(* Logix 5000 AddOnInstructionDefinition export Banner_TL70Pro_Param_v4; software revision 33.00 *)

TYPE Banner_IOL_Port_v4 :   // UDT that has all of the data items necessary to communicate with a specific Port on a IO-Link Master
STRUCT
   Port_Controlled : INT;   // Each bit represents a port on an IO-Link Master. Set to 1 to tell AOI to control that port.
   Port_Activate : INT;   // Each bit represents a port on an IO-Link Master. When ON that port will process any commands in queue.
   Port_Read : INT;   // Each bit represents a port on an IO-Link Master. Used to determine when device AOI has requested a Read command.
   Port_Write : INT;   // Each bit represents a port on an IO-Link Master. Used to determine when device AOI has requested a Write command.
   Port_RW_Complete : INT;   // Each bit represents a port on an IO-Link Master. Tells device AOI that Read or Write request has been completed.
   Port_Device_Read : INT;
   Data_Transfer : SINT[190];   // Array to transfer data from IO-Master to device AOIs.
END_STRUCT
END_TYPE

TYPE Banner_TL70Pro_Basic_SP_v4 :   // Basic parameters for a TL70 Pro segment.
STRUCT
   Basic_Color : SINT;   // 0 = Green, 1 = Red, 2 = Orange, 3 = Amber, 4 = Yellow, 5 = Lime Green, 6 = Spring Green, 7 = Cyan, 8 = Sky Blue, 9 = Blue, 10 = Violet, 11 = Magenta, 12 = Rose, 13 = White, 14 = Custom, 15 = Custom 2
   Basic_Flash_Rate : SINT;   // 0 = Medium, 1 = Fast, 2 = Slow, 3 = Custom Flash Rate
   Animation : SINT;   // 0 = Off, 1 = Steady, 2 = Flash, 3 = Two Color, 4 = Half/Half, 5 = Half/Half Rotate, 6 = Chase, 7 = Intesnity Sweep
   Color_1 : INT;   // 0 = Green, 1 = Red, 2 = Orange, 3 = Amber, 4 = Yellow, 5 = Lime Green, 6 = Spring Green, 7 = Cyan, 8 = Sky Blue, 9 = Blue, 10 = Violet, 11 = Magenta, 12 = Rose, 13 = White, 14 = Custom, 15 = Custom 2
   Color_1_Intensity : SINT;   // 0 = High, 1 = Low, 2 = Medium, 3 = Off, 4 = Custom
   Speed : SINT;   // 0 = Medium, 1 = Fast, 2 = Slow, 3 = Custom
   Pulse_Pattern : SINT;   // 0 = Normal, 1 = Strobe, 2 = Three Pulse, 3 = SOS, 4 = Random
   Color_2 : SINT;   // 0 = Green, 1 = Red, 2 = Orange, 3 = Amber, 4 = Yellow, 5 = Lime Green, 6 = Spring Green, 7 = Cyan, 8 = Sky Blue, 9 = Blue, 10 = Violet, 11 = Magenta, 12 = Rose, 13 = White, 14 = Custom, 15 = Custom 2
   Color_2_Intensity : SINT;   // 0 = High, 1 = Low, 2 = Medium, 3 = Off, 4 = Custom
END_STRUCT
END_TYPE

TYPE Banner_TL70Pro_Gauge_Center_Settings_v4 :   // TL70 Pro. BG = Background
STRUCT
   Percent_Width_of_Main_Segment : SINT;   // 1 to 100
   Main_Animation : INT;   // 0 = Off, 1 = Steady, 2 = Flash, 3 = Two Color Flash, 4 = Two Color Shift, 5 = Scroll, 6 = Center Scroll, 7 = Bounce, 8 = Center Bounce, 9 = Intensity Sweep, 10 = Two Color Sweep, 11 = Spectrum, 12 = Single End Steady, 13 = Single End Flash
   Main_Color_1 : INT;   // 0 = Green, 1 = Red, 2 = Orange, 3 = Amber, 4 = Yellow, 5 = Lime Green, 6 = Spring Green, 7 = Cyan, 8 = Sky Blue, 9 = Blue, 10 = Violet, 11 = Magenta, 12 = Rose, 13 = White, 14 = Custom, 15 = Custom 2
   Main_Color_1_Intensity : SINT;   // 0 = High, 1 = Low, 2 = Medium, 3 = Off, 4 = Custom
   Main_Speed : SINT;   // 0 = Medium, 1 = Fast, 2 = Slow, 3 = Custom Flash Rate
   Main_Pulse_Pattern : SINT;   // 0 = Normal, 1 = Strobe, 2 = Three Pulse, 3 = SOS, 4 = Random
   Main_Color_2 : INT;   // 0 = Green, 1 = Red, 2 = Orange, 3 = Amber, 4 = Yellow, 5 = Lime Green, 6 = Spring Green, 7 = Cyan, 8 = Sky Blue, 9 = Blue, 10 = Violet, 11 = Magenta, 12 = Rose, 13 = White, 14 = Custom, 15 = Custom 2
   Main_Color_2_Intensity : SINT;   // 0 = High, 1 = Low, 2 = Medium, 3 = Off, 4 = Custom
   Main_Scroll_Bounce_Style : SINT;   // 0 = Solid,1 = Tail, 2 = Ripple
   Main_Percent_Width_of_Color_1 : SINT;   // 0 to 100
   Main_Direction : SINT;   // 0 = Up, 1 = Down
   BG_Animation : INT;   // 0 = Off, 1 = Steady, 2 = Flash, 3 = Two Color Flash, 4 = Two Color Shift, 5 = Scroll, 6 = Center Scroll, 7 = Bounce, 8 = Center Bounce, 9 = Intensity Sweep, 10 = Two Color Sweep, 11 = Spectrum, 12 = Single End Steady, 13 = Single End Flash
   BG_Color_1 : INT;   // 0 = Green, 1 = Red, 2 = Orange, 3 = Amber, 4 = Yellow, 5 = Lime Green, 6 = Spring Green, 7 = Cyan, 8 = Sky Blue, 9 = Blue, 10 = Violet, 11 = Magenta, 12 = Rose, 13 = White, 14 = Custom, 15 = Custom 2
   BG_Color_1_Intensity : INT;   // 0 = High, 1 = Low, 2 = Medium, 3 = Off, 4 = Custom
   BG_Speed : SINT;   // 0 = Medium, 1 = Fast, 2 = Slow, 3 = Custom
   BG_Pulse_Pattern : SINT;   // 0 = Normal, 1 = Strobe, 2 = Three Pulse, 3 = SOS, 4 = Random
   BG_Color_2 : INT;   // 0 = Green, 1 = Red, 2 = Orange, 3 = Amber, 4 = Yellow, 5 = Lime Green, 6 = Spring Green, 7 = Cyan, 8 = Sky Blue, 9 = Blue, 10 = Violet, 11 = Magenta, 12 = Rose, 13 = White, 14 = Custom, 15 = Custom 2
   BG_Color_2_Intensity : SINT;   // 0 = High, 1 = Low, 2 = Medium, 3 = Off, 4 = Custom
   BG_Scroll_Bounce_Style : SINT;   // 0 = Solid, 1 = Tail, 2 = Ripple
   BG_Percent_Width_of_Color_1 : SINT;   // 1 to 100
   BG_Direction : SINT;   // 0 = Up, 1 = Down
END_STRUCT
END_TYPE

TYPE Banner_TL70Pro_Gauge_Mode_Config_v4 :
STRUCT
   Filtering : SINT;   // 0 = None, 1 = Low, 2 = Medium, 3 = High
   Hysteresis : SINT;   // 0 = None, 1 = Low, 2 = Medium, 3 = High
   Full_Scale_Value : INT;   // 0 to 100
END_STRUCT
END_TYPE

TYPE Banner_TL70Pro_Gauge_Threshold_Set_v4 :   // BG = Background
STRUCT
   Threshold_Enable : SINT;   // 0 = Threshold Disabled, 1 = Threshold Enabled
   Threshold_Value : SINT;   // 0 to 100 percent
   Threshold_Comparison : SINT;   // 0 = Less than or equal to, 1 = Greater than or equal to
   Percent_Width_of_Main_Segment : SINT;   // 0 to 100 percent
   Main_Animation : INT;   // 0 = Off, 1 = Steady, 2 = Flash, 3 = Two Color Flash, 4 = Two Color Shift, 5 = Scroll, 6 = Center Scroll, 7 = Bounce, 8 = Center Bounce, 9 = Intensity Sweep, 10 = Two Color Sweep, 11 = Spectrum, 12 = Single End Steady, 13 = Single End Flash
   Main_Color_1 : INT;   // 0 = Green, 1 = Red, 2 = Orange, 3 = Amber, 4 = Yellow, 5 = Lime Green, 6 = Spring Green, 7 = Cyan, 8 = Sky Blue, 9 = Blue, 10 = Violet, 11 = Magenta, 12 = Rose, 13 = White, 14 = Custom, 15 = Custom 2
   Main_Color_1_Intensity : SINT;   // 0 = High, 1= Low, 2 = Medium, 3 = Off, 4 = Custom
   Main_Speed : SINT;   // 0 = Medium, 1 = Fast, 2 = Slow, 3 = Custom Flash Rate
   Main_Pulse_Pattern : SINT;   // 0 = Normal, 1 = Strobe, 2 = Three Pulse, 3 = SOS, 4 = Random
   Main_Color_2 : INT;   // 0 = Green, 1 = Red, 2 = Orange, 3 = Amber, 4 = Yellow, 5 = Lime Green, 6 = Spring Green, 7 = Cyan, 8 = Sky Blue, 9 = Blue, 10 = Violet, 11 = Magenta, 12 = Rose, 13 = White, 14 = Custom, 15 = Custom 2
   Main_Color_2_Intensity : SINT;   // 0 = High,1 = Low, 2= Medium, 3 = Off, 4 = Custom
   Main_Scroll_Bounce_Style : SINT;   // 0 = Solid, 1 = Tail, 2 = Ripple
   Main_Percent_Width_of_Color_1 : SINT;   // 1 to 100 percent
   Main_Direction : SINT;   // 0 = Up, 1 = Down
   BG_Animation : INT;   // 0 = Off, 1 = Steady, 2 = Flash, 3 = Two Color Flash, 4 = Two Color Shift, 5 = Scroll, 6 = Center Scroll, 7 = Bounce, 8 = Center Bounce, 9 = Intensity Sweep, 10 = Two Color Sweep, 11 = Spectrum, 12 = Single End Steady, 13 = Single End Flash
   BG_Color_1 : INT;   // 0 = Green, 1 = Red, 2 = Orange, 3 = Amber, 4 = Yellow, 5 = Lime Green, 6 = Spring Green, 7 = Cyan, 8 = Sky Blue, 9 = Blue, 10 = Violet, 11 = Magenta, 12 = Rose, 13 = White, 14 = Custom, 15 = Custom 2
   BG_Color_1_Intensity : SINT;   // 0 = High, 1 = Low, 2 = Medium, 3 = Off, 4 = Custom
   BG_Speed : SINT;   // 0 = Medium, 1 = Fast, 2 = Slow, 3 = Custom Flash Rate
   BG_Pulse_Pattern : SINT;   // 0 = Normal, 1 = Strobe, 2 = Three Pulse, 3 = SOS, 4 = Random
   BG_Color_2 : INT;   // 0 = Green, 1 = Red, 2 = Orange, 3 = Amber, 4 = Yellow, 5 = Lime Green, 6 = Spring Green, 7 = Cyan, 8 = Sky Blue, 9 = Blue, 10 = Violet, 11 = Magenta, 12 = Rose, 13 = White, 14 = Custom, 15 = Custom 2
   BG_Color_2_Intensity : SINT;   // 0 = High, 1 = Low, 2 = Medium, 3 = Off, 4 = Custom
   BG_Scroll_Bounce_Style : SINT;   // 0 = Solid, 1 = Tail, 2 = Ripple
   BG_Percent_Width_of_Color_1 : SINT;   // 1 to 100
   BG_Direction : SINT;   // 0 = Up, 1 = Down
END_STRUCT
END_TYPE

TYPE Banner_TL70Pro_General_Level_Config_v4 :
STRUCT
   BG_Color : SINT;   // Background Color. 0 = Green, 1 = Red, 2 = Orange, 3 = Amber, 4 = Yellow, 5 = Lime Green, 6 = Spring Green, 7 = Cyan, 8 = Sky Blue, 9 = Blue, 10 = Violet, 11 = Magenta, 12 = Rose, 13 = White, 14 = Custom, 15 = Custom 2.
   BG_Intensity : SINT;   // 0 = High, 1 = Low, 2 = Medium, 3 = Off, 4 = Custom
   Dominance : SINT;   // 0 = Non-Dominant, 1 = Dominant
   Sub_Segment_Style : SINT;   // 0 = Solid, 1 = Analog
   Filtering : SINT;   // 0 = None, 1 = Low, 2 = Medium, 3 = High
   Hysteresis : SINT;   // 0 = None, 1 = Low, 2 = Medium, 3 = High
   Full_Scale_Value : INT;
END_STRUCT
END_TYPE

TYPE Banner_TL70Pro_General_Seg_Config_v4 :
STRUCT
   Background_Color : INT;   // 0 = Green, 1 = Red, 2 = Orange, 3 = Amber, 4 = Yellow, 5 = Lime Green, 6 = Spring Green, 7 = Cyan, 8 = Sky Blue, 9 = Blue, 10 = Violet, 11 = Magenta, 12 = Rose, 13 = White, 14 = Custom, 15 = Custom 2
   Background_Intensity : SINT;   // 0 = High, 1 = Low, 2 = Medium, 3 = Off, 4 = Custom
   Animation_Synchro : SINT;   // 0 = Animation Sync Disabled, 1 = Animation Sync Enabled
END_STRUCT
END_TYPE

TYPE Banner_TL70Pro_Level_Base_Config_v4 :
STRUCT
   Animation : INT;   // 0 = Off, 1 = Steady, 2 = Flash, 3 = Two Color Flash, 4 = Two Color Shift, 5 = Scroll, 6 = Center Scroll, 7 = Bounce, 8 = Center Bounce, 9 = Intensity Sweep, 10 = Two Color Sweep, 11 = Spectrum, 12 = Single End Steady, 13 = Daylight White, 14 = Custom 1, 15 = Custom 2
   Color_1 : INT;   // 0 = Green, 1 = Red, 2 = Orange, 3 = Amber, 4 = Yellow, 5 = Lime Green, 6 = Spring Green, 7 = Cyan, 8 = Sky Blue, 9 = Blue, 10 = Violet, 11 = Magenta, 12 = Rose, 13 = White, 14 = Custom, 15 = Custom 2
   Color_1_Intensity : SINT;   // 0 = High, 1 = Low, 2 = Medium, 3 = Off, 4 = Custom
   Speed : SINT;   // 0 = Medium, 1 = Fast, 2 = Slow, 3 = Custom Flash Rate
   Pulse_Pattern : SINT;   // 0 = Normal, 1 = Strobe, 2 = Three Pulse, 3 = SOS, 4 = Random
   Color_2 : INT;   // 0 = Green, 1 = Red, 2 = Orange, 3 = Amber, 4 = Yellow, 5 = Lime Green, 6 = Spring Green, 7 = Cyan, 8 = Sky Blue, 9 = Blue, 10 = Violet, 11 = Magenta, 12 = Rose, 13 = White, 14 = Custom, 15 = Custom 2
   Color_2_Intensity : INT;   // 0 = High, 1 = Low, 2 = Medium, 3 = Off, 4 = Custom
   Scroll_Bounce_Style : SINT;   // 0 = Solid, 1 = Tail, 2 = Ripple
   Percent_Width_of_Color_1 : SINT;   // 0 to 100. The size of the scrolling segement
   Direction : SINT;   // 0 = Up, 1 = Down
END_STRUCT
END_TYPE

TYPE Banner_TL70Pro_RD_v4 :   // UDT that stores the Read Data for a TL70 Pro.
STRUCT
   Master_Cycle_Time : INT;
   Min_Cycle_Time : INT;
   M_Sequence_Capability : INT;
   IO_Link_Version_ID : INT;
   Process_Data_Input_Length : INT;
   Process_Data_Output_Length : INT;
   Combined_Vendor_ID : DINT;   // IO-Link Vendor ID
   Vendor_ID1 : INT;
   Vendor_ID2 : INT;
   Combined_Device_ID : DINT;   // IO-Link Device ID
   Device_ID1 : INT;
   Device_ID2 : INT;
   Device_ID3 : INT;
   Serial_Number : STRING;
END_STRUCT
END_TYPE

TYPE Banner_TL70Pro_Threshold_Config_v4 :
STRUCT
   Threshold_Enable : SINT;   // 0 = Threshold Disabled, 1 = Threshold Enabled
   Threshold_Value_Percent : SINT;   // 0 to 100 percent.
   Threshold_Comparison : SINT;   // 0 = Less than or equal to, 1 = Greater than or equal to
   Threshold_Override : SINT;   // 0 = Override not enabled, 1 = Override Enabled
   Animation : INT;   // 0 = Off, 1 = Steady, 2 = Flash, 3 = Two Color Flash, 4 = Two Color Shift, 5 = Scroll, 6 = Center Scroll, 7 = Bounce, 8 = Center Bounce, 9 = Intensity Sweep, 10 = Two Color Sweep, 11 = Spectrum, 12 = Single End Steady, 13 = Single End Flash
   Color_1 : INT;   // 0 = Green, 1 = Red, 2 = Orange, 3 = Amber, 4 = Yellow, 5 = Lime Green, 6 = Spring Green, 7 = Cyan, 8 = Sky Blue, 9 = Blue, 10 = Violet, 11 = Magenta, 12 = Rose, 13 = White, 14 = Custom, 15 = Custom 2
   Color_1_Intensity : SINT;   // 0 = High, 1 = Low, 2 = Medium, 3 = Off, 4 = Custom
   Speed : SINT;   // 0 = Medium, 1 = Fast, 2 = Slow, 3 = Custom Flash Rate
   Pulse_Pattern : SINT;   // 0 = Normal, 1 = Strobe, 2 = Three Pulse, 3 = SOS, 4 = Random
   Color_2 : INT;   // 0 = Green, 1 = Red, 2 = Orange, 3 = Amber, 4 = Yellow, 5 = Lime Green, 6 = Spring Green, 7 = Cyan, 8 = Sky Blue, 9 = Blue, 10 = Violet, 11 = Magenta, 12 = Rose, 13 = White, 14 = Custom, 15 = Custom 2
   Color_2_Intensity : SINT;   // 0 = High, 1 = Low, 2 = Medium, 3 = Off, 4 = Custom
   Scroll_Bounce_Style : SINT;   // 0 = Solid, 1 = Tail, 2 = Ripple
   Percent_Width_of_Color_1 : SINT;   // 0 to 100
   Direction : SINT;   // 0 = Up, 1 = Down
END_STRUCT
END_TYPE

TYPE Banner_TL70Pro_v4 :   // All of the parameters for a TL70 Pro.
STRUCT
   Initial_Global_Read : BOOL;   // Determines if all of the IO-Link data has been read into the PLC yet
   Command : INT;   // Value placed in here will activate a read or write to a specifc IO-Link Index
   Read : Banner_TL70Pro_RD_v4;   // Read Only Data
   Write : Banner_TL70Pro_WD_v4;   // Write Data
   Archive : Banner_TL70Pro_WD_v4;   // Archive of the Write Data
   Reset : BOOL;   // Resets AOI. This will force a complete parameter read of the sensor.
END_STRUCT
END_TYPE

TYPE Banner_TL70Pro_WD_v4 :   // UDT that stores the Write Data for a TL70 Pro.
STRUCT
   System_Command : INT;   // See IODD file for list of commands that can be activated via the System Command interface
   Parameter_Access_Lock : SINT;   // Write access to all parameters is prohibited while value is 1. Only this parameter can be adjusted when value is 1.
   Data_Storage_Lock : SINT;   // Automatic data storage is disabled when this value is equal to 1. Read access is not affected.
   Local_Parameterization_Lock : SINT;   // Parameterization via local control elements on device is disabled.
   Local_User_Interface_Lock : SINT;   // Operation of local user interface is disabled.
   Operating_Mode_Selection : SINT;   // 0 = Basic Mode, 1 = Run Mode, 2 = Level Mode, 3 = Gauge Mode, 4 = Advance Mode
   General_Segment_Config : Banner_TL70Pro_General_Seg_Config_v4;
   Segment_Config : Banner_TL70Pro_Basic_SP_v4[7];
   General_Level_Config : Banner_TL70Pro_General_Level_Config_v4;
   Level_Base_Config : Banner_TL70Pro_Level_Base_Config_v4;
   Level_Threshold_Config : Banner_TL70Pro_Threshold_Config_v4[5];
   Custom_1_Red : INT;   // 0 to 255. Value of the Red portion of the RGB color value for Custom 1
   Custom_1_Green : INT;   // 0 to 255. Value of the Green portion of the RGB color value for Custom 1.
   Custom_1_Blue : INT;   // 0 to 255. Value of the Blue portion of the RGB color value for Custom 1.
   Custom_2_Red : INT;   // 0 to 255. Value of the Red portion of the RGB color value for Custom 2.
   Custom_2_Green : INT;   // 0 to 255. Value of the Green portion of the RGB color value for Custom 2.
   Custom_2_Blue : INT;   // 0 to 255. Value of the Blue portion of the RGB color value for Custom 2.
   Orientation : SINT;   // 0 = Standard, 1 = Inverted
   Custom_Intensity : SINT;   // 0 to 100
   Custom_Frequency : INT;   // 0 to 255
   Gauge_Mode_Config : Banner_TL70Pro_Gauge_Mode_Config_v4;
   Gauge_Mode_Center : Banner_TL70Pro_Gauge_Center_Settings_v4;
   Gauge_Mode_Threshold : Banner_TL70Pro_Gauge_Threshold_Set_v4[3];
   Advanced_Audible_Type : SINT;   // 0 = Beep, 1 = Sweep, 2 = Tone
   Sweep_Type : SINT;   // 0 = Up, 1 = Down, 2 = Up Down, 3 = Down Up
   Frequency_1 : SINT;   // 0 = Off, 1 = Low, 2 = Standard, 3 = High
   Frequency_2 : SINT;   // 0 = Off, 1 = Low, 2 = Standard, 3 = High
END_STRUCT
END_TYPE

ADD_ON_INSTRUCTION Banner_TL70Pro_Param_v4   (* revision 4.1, vendor Banner Engineering *)
// AOI to read and write parameter data to an IO-Link TL70 Pro.
VAR_IN_OUT
   TL70Pro : Banner_TL70Pro_v4; {required}
   Port_Data : Banner_IOL_Port_v4; {required}
END_VAR
VAR_INPUT
   Port : INT; {required}   // Port Number that device is plugged into.
END_VAR
VAR
   Local_Control : DINT; {access None}
   Global_Read_Command_Value : INT; {access None}
   Global_Write_Command_Value : INT; {access None}
   Command_Being_Processed : BOOL; {access None}
   Update_Archive : BOOL; {access None}
   Index_Write_Inprocess : DINT; {access None}
   Index_Write_Control : DINT; {access None}
   Inprocess_Index : DINT; {access None}
   Index_R : DINT; {access None}
   BS_Index : DINT; {access None}
   Index_W : DINT; {access None}
   W_Index : DINT; {access None}
   Index_Segment_Read : DINT; {access None}
   GT_Index2 : DINT; {access None}
   GT_Index1 : DINT; {access None}
   LT_Index2 : DINT; {access None}
   LT_Index1 : DINT; {access None}
END_VAR

ROUTINE Logic   (* ladder *)
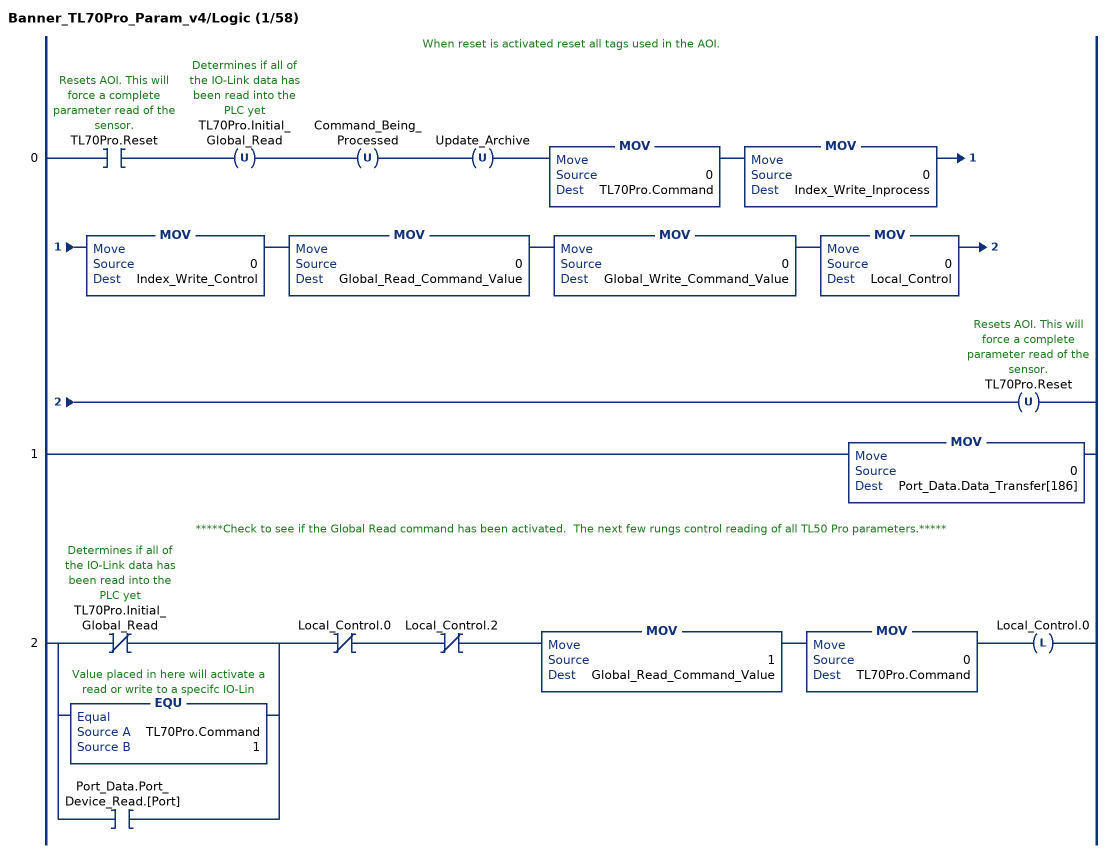
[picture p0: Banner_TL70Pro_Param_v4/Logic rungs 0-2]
   // When reset is activated reset all tags used in the AOI.
   0: XIC(TL70Pro.Reset)OTU(TL70Pro.Initial_Global_Read)OTU(Command_Being_Processed)OTU(Update_Archive)MOV(0,TL70Pro.Command)MOV(0,Index_Write_Inprocess)MOV(0,Index_Write_Control)MOV(0,Global_Read_Command_Value)MOV(0,Global_Write_Command_Value)MOV(0,Local_Control)OTU(TL70Pro.Reset);
   1: MOV(0,Port_Data.Data_Transfer[186]);
   // *****Check to see if the Global Read command has been activated.  The next few rungs control reading of all TL50 Pro parameters.*****
   2: [XIO(TL70Pro.Initial_Global_Read) ,EQU(TL70Pro.Command,1) ,XIC(Port_Data.Port_Device_Read.[Port]) ]XIO(Local_Control.0)XIO(Local_Control.2)MOV(1,Global_Read_Command_Value)MOV(0,TL70Pro.Command)OTL(Local_Control.0);
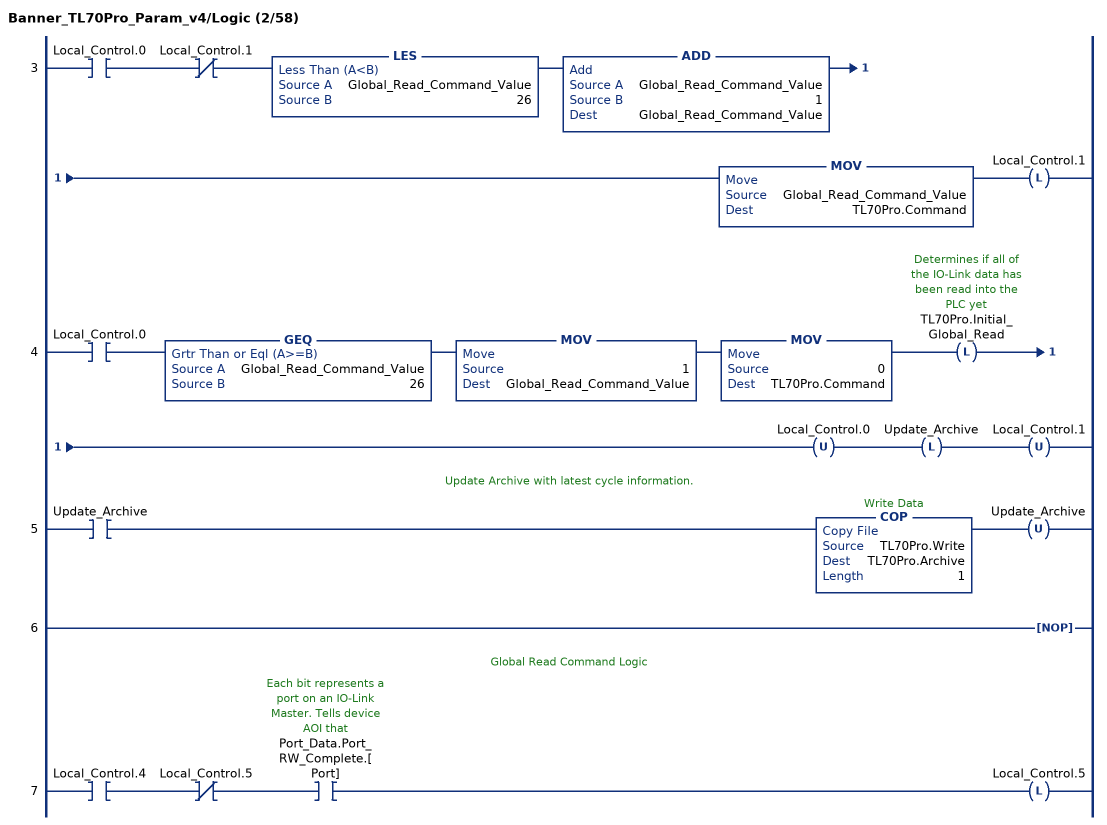
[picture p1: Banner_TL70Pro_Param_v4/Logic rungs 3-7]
   3: XIC(Local_Control.0)XIO(Local_Control.1)LES(Global_Read_Command_Value,26)ADD(Global_Read_Command_Value,1,Global_Read_Command_Value)MOV(Global_Read_Command_Value,TL70Pro.Command)OTL(Local_Control.1);
   4: XIC(Local_Control.0)GEQ(Global_Read_Command_Value,26)MOV(1,Global_Read_Command_Value)MOV(0,TL70Pro.Command)OTL(TL70Pro.Initial_Global_Read)OTU(Local_Control.0)OTL(Update_Archive)OTU(Local_Control.1);
   // Update Archive with latest cycle information.
   5: XIC(Update_Archive)COP(TL70Pro.Write,TL70Pro.Archive,1)OTU(Update_Archive);
   6: NOP();
   // Global Read Command Logic
   7: XIC(Local_Control.4)XIO(Local_Control.5)XIC(Port_Data.Port_RW_Complete.[Port])OTL(Local_Control.5);
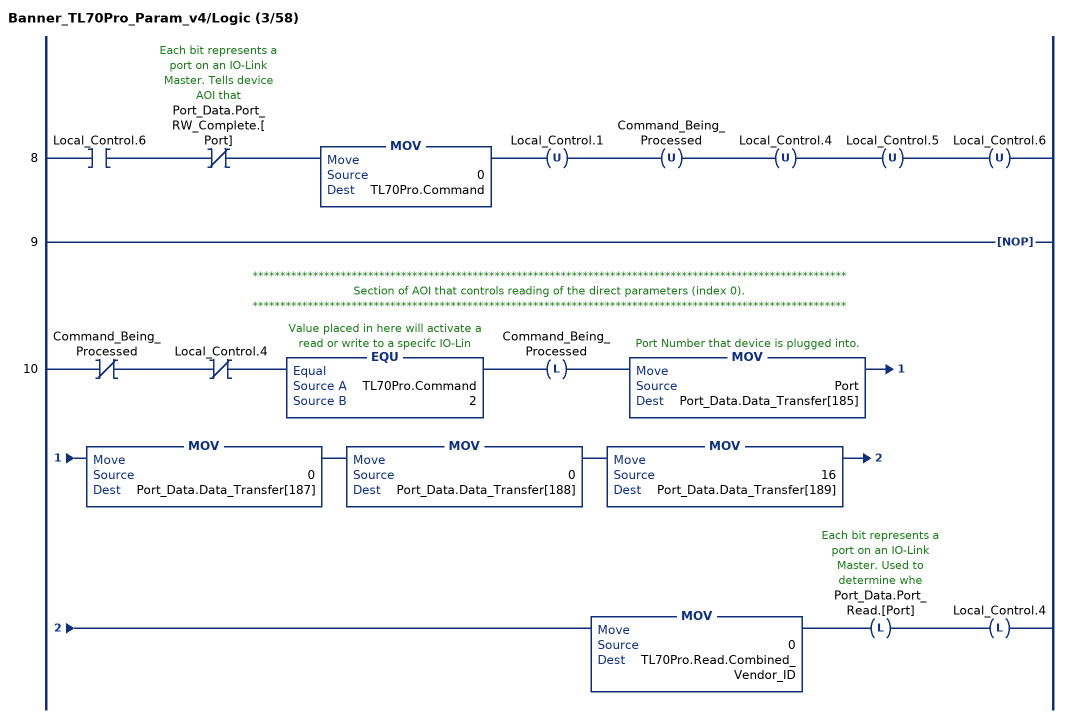
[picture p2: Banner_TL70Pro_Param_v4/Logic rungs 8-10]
   8: XIC(Local_Control.6)XIO(Port_Data.Port_RW_Complete.[Port])MOV(0,TL70Pro.Command)OTU(Local_Control.1)OTU(Command_Being_Processed)OTU(Local_Control.4)OTU(Local_Control.5)OTU(Local_Control.6);
   9: NOP();
   // ************************************************************************************************************
   // Section of AOI that controls reading of the direct parameters (index 0).
   // ************************************************************************************************************
   10: XIO(Command_Being_Processed)XIO(Local_Control.4)EQU(TL70Pro.Command,2)OTL(Command_Being_Processed)MOV(Port,Port_Data.Data_Transfer[185])MOV(0,Port_Data.Data_Transfer[187])MOV(0,Port_Data.Data_Transfer[188])MOV(16,Port_Data.Data_Transfer[189])MOV(0,TL70Pro.Read.Combined_Vendor_ID)OTL(Port_Data.Port_Read.[Port])OTL(Local_Control.4);
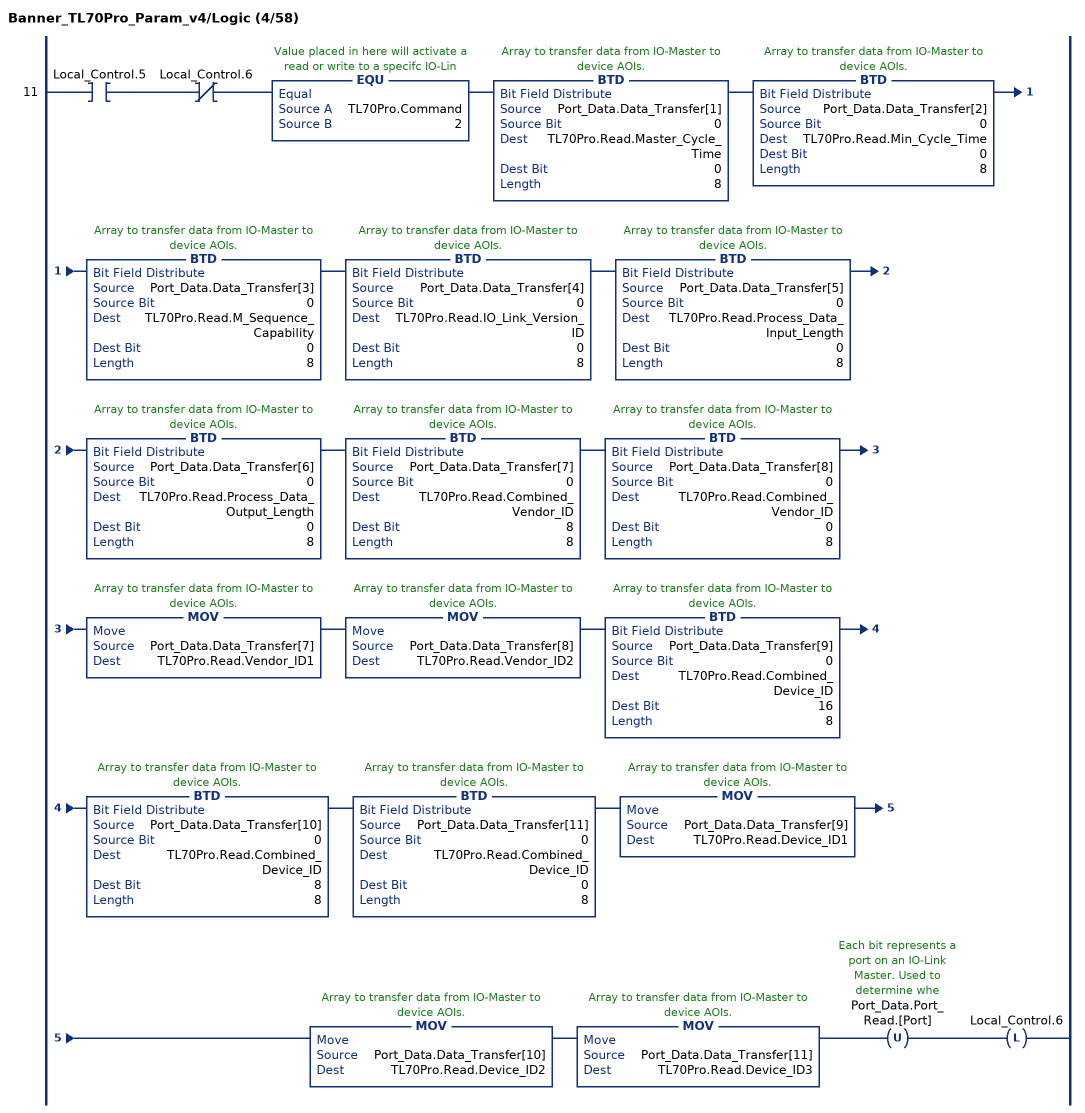
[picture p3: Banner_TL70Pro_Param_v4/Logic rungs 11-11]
   11: XIC(Local_Control.5)XIO(Local_Control.6)EQU(TL70Pro.Command,2)BTD(Port_Data.Data_Transfer[1],0,TL70Pro.Read.Master_Cycle_Time,0,8)BTD(Port_Data.Data_Transfer[2],0,TL70Pro.Read.Min_Cycle_Time,0,8)BTD(Port_Data.Data_Transfer[3],0,TL70Pro.Read.M_Sequence_Capability,0,8)BTD(Port_Data.Data_Transfer[4],0,TL70Pro.Read.IO_Link_Version_ID,0,8)BTD(Port_Data.Data_Transfer[5],0,TL70Pro.Read.Process_Data_Input_Length,0,8)BTD(Port_Data.Data_Transfer[6],0,TL70Pro.Read.Process_Data_Output_Length,0,8)BTD(Port_Data.Data_Transfer[7],0,TL70Pro.Read.Combined_Vendor_ID,8,8)BTD(Port_Data.Data_Transfer[8],0,TL70Pro.Read.Combined_Vendor_ID,0,8)MOV(Port_Data.Data_Transfer[7],TL70Pro.Read.Vendor_ID1)MOV(Port_Data.Data_Transfer[8],TL70Pro.Read.Vendor_ID2)BTD(Port_Data.Data_Transfer[9],0,TL70Pro.Read.Combined_Device_ID,16,8)BTD(Port_Data.Data_Transfer[10],0,TL70Pro.Read.Combined_Device_ID,8,8)BTD(Port_Data.Data_Transfer[11],0,TL70Pro.Read.Combined_Device_ID,0,8)MOV(Port_Data.Data_Transfer[9],TL70Pro.Read.Device_ID1)MOV(Port_Data.Data_Transfer[10],TL70Pro.Read.Device_ID2)MOV(Port_Data.Data_Transfer[11],TL70Pro.Read.Device_ID3)OTU(Port_Data.Port_Read.[Port])OTL(Local_Control.6);
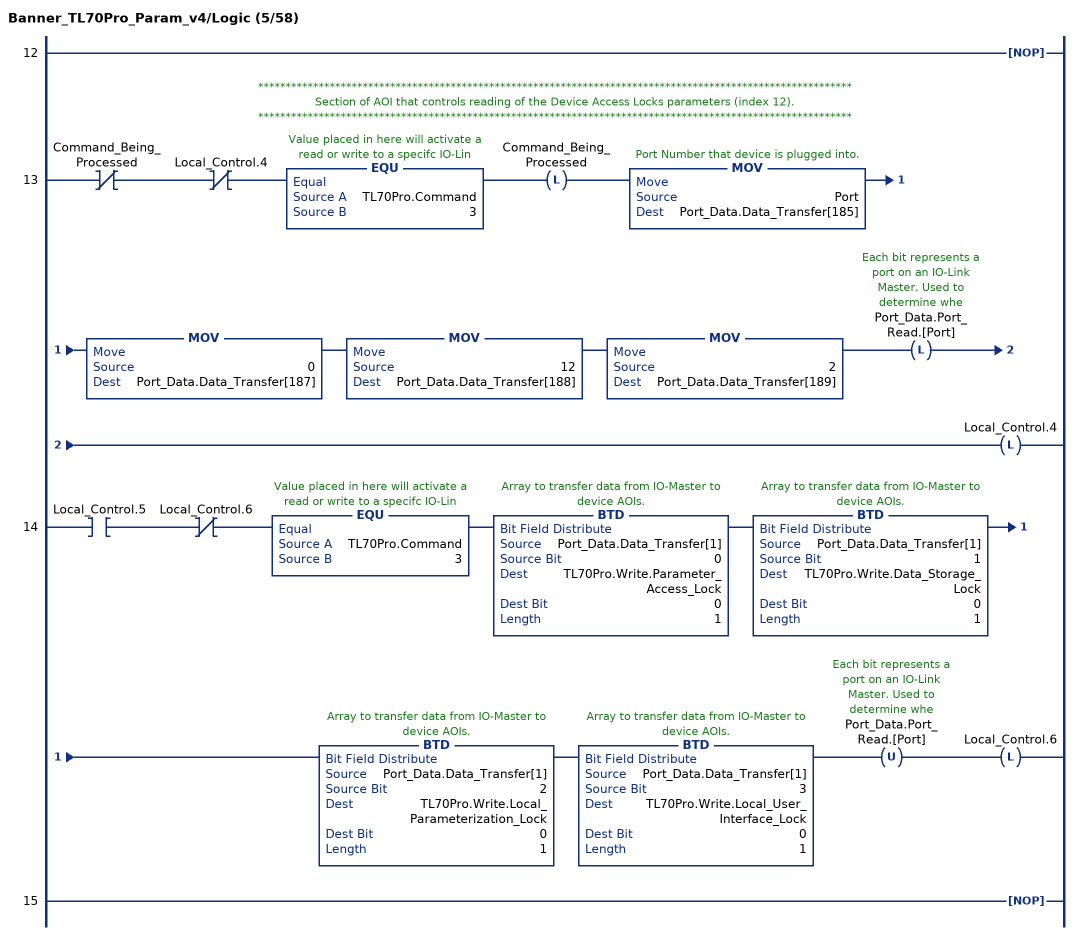
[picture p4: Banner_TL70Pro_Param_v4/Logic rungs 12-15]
   12: NOP();
   // ************************************************************************************************************
   // Section of AOI that controls reading of the Device Access Locks parameters (index 12).
   // ************************************************************************************************************
   13: XIO(Command_Being_Processed)XIO(Local_Control.4)EQU(TL70Pro.Command,3)OTL(Command_Being_Processed)MOV(Port,Port_Data.Data_Transfer[185])MOV(0,Port_Data.Data_Transfer[187])MOV(12,Port_Data.Data_Transfer[188])MOV(2,Port_Data.Data_Transfer[189])OTL(Port_Data.Port_Read.[Port])OTL(Local_Control.4);
   14: XIC(Local_Control.5)XIO(Local_Control.6)EQU(TL70Pro.Command,3)BTD(Port_Data.Data_Transfer[1],0,TL70Pro.Write.Parameter_Access_Lock,0,1)BTD(Port_Data.Data_Transfer[1],1,TL70Pro.Write.Data_Storage_Lock,0,1)BTD(Port_Data.Data_Transfer[1],2,TL70Pro.Write.Local_Parameterization_Lock,0,1)BTD(Port_Data.Data_Transfer[1],3,TL70Pro.Write.Local_User_Interface_Lock,0,1)OTU(Port_Data.Port_Read.[Port])OTL(Local_Control.6);
   15: NOP();
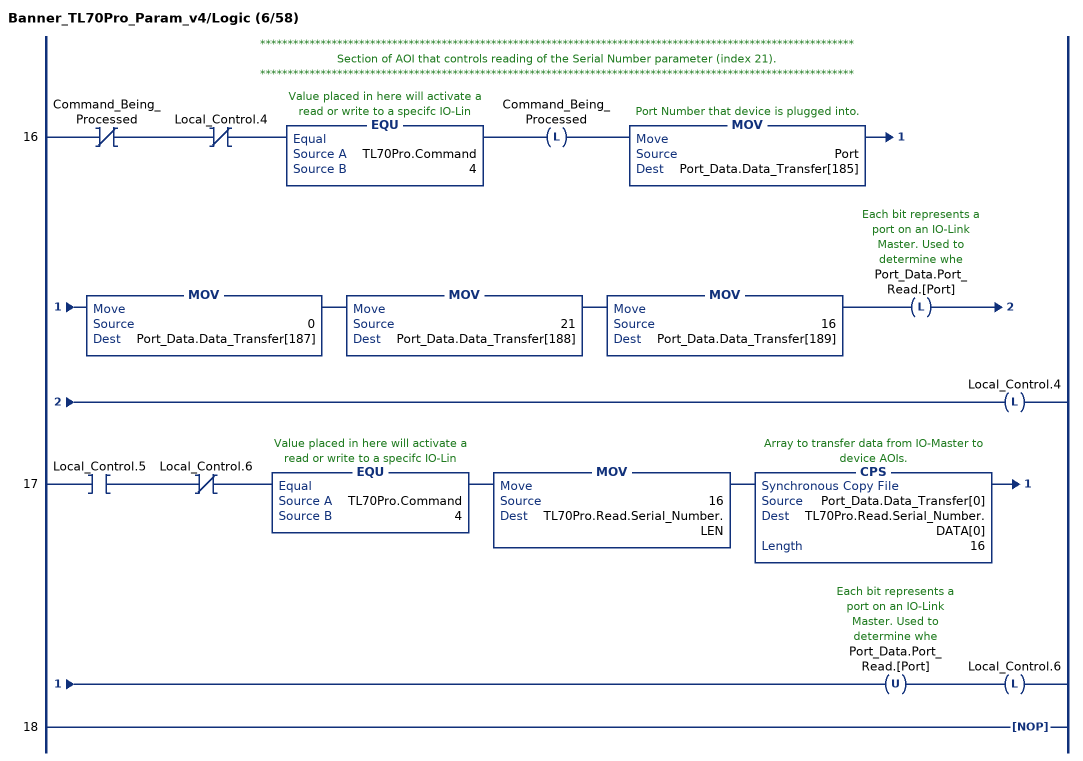
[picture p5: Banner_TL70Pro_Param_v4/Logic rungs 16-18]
   // ************************************************************************************************************
   // Section of AOI that controls reading of the Serial Number parameter (index 21).
   // ************************************************************************************************************
   16: XIO(Command_Being_Processed)XIO(Local_Control.4)EQU(TL70Pro.Command,4)OTL(Command_Being_Processed)MOV(Port,Port_Data.Data_Transfer[185])MOV(0,Port_Data.Data_Transfer[187])MOV(21,Port_Data.Data_Transfer[188])MOV(16,Port_Data.Data_Transfer[189])OTL(Port_Data.Port_Read.[Port])OTL(Local_Control.4);
   17: XIC(Local_Control.5)XIO(Local_Control.6)EQU(TL70Pro.Command,4)MOV(16,TL70Pro.Read.Serial_Number.LEN)CPS(Port_Data.Data_Transfer[0],TL70Pro.Read.Serial_Number.DATA[0],16)OTU(Port_Data.Port_Read.[Port])OTL(Local_Control.6);
   18: NOP();
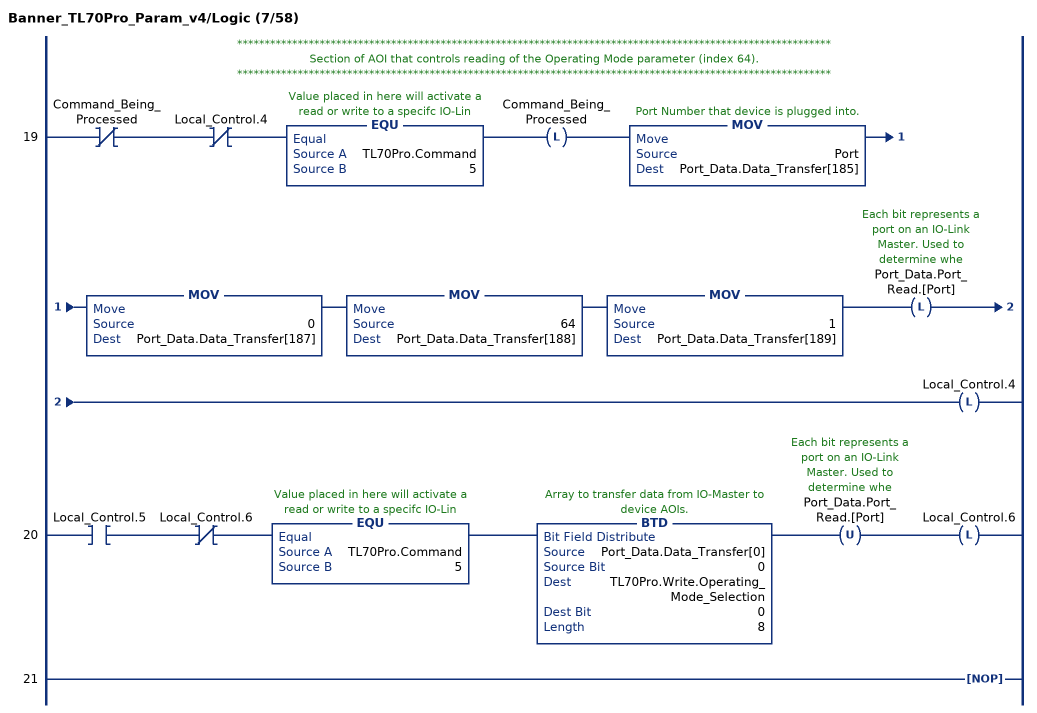
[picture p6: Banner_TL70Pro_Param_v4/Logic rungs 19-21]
   // ************************************************************************************************************
   // Section of AOI that controls reading of the Operating Mode parameter (index 64).
   // ************************************************************************************************************
   19: XIO(Command_Being_Processed)XIO(Local_Control.4)EQU(TL70Pro.Command,5)OTL(Command_Being_Processed)MOV(Port,Port_Data.Data_Transfer[185])MOV(0,Port_Data.Data_Transfer[187])MOV(64,Port_Data.Data_Transfer[188])MOV(1,Port_Data.Data_Transfer[189])OTL(Port_Data.Port_Read.[Port])OTL(Local_Control.4);
   20: XIC(Local_Control.5)XIO(Local_Control.6)EQU(TL70Pro.Command,5)BTD(Port_Data.Data_Transfer[0],0,TL70Pro.Write.Operating_Mode_Selection,0,8)OTU(Port_Data.Port_Read.[Port])OTL(Local_Control.6);
   21: NOP();
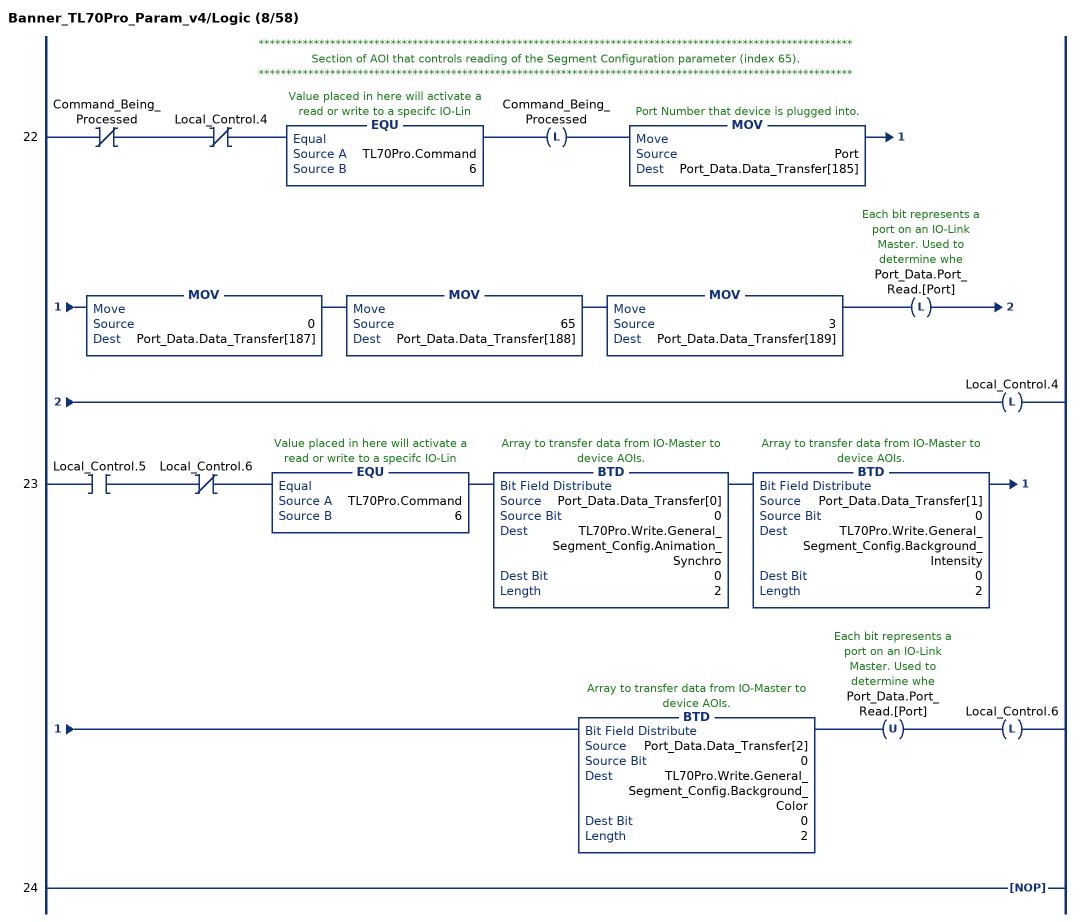
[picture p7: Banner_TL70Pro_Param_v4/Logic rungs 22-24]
   // ************************************************************************************************************
   // Section of AOI that controls reading of the Segment Configuration parameter (index 65).
   // ************************************************************************************************************
   22: XIO(Command_Being_Processed)XIO(Local_Control.4)EQU(TL70Pro.Command,6)OTL(Command_Being_Processed)MOV(Port,Port_Data.Data_Transfer[185])MOV(0,Port_Data.Data_Transfer[187])MOV(65,Port_Data.Data_Transfer[188])MOV(3,Port_Data.Data_Transfer[189])OTL(Port_Data.Port_Read.[Port])OTL(Local_Control.4);
   23: XIC(Local_Control.5)XIO(Local_Control.6)EQU(TL70Pro.Command,6)BTD(Port_Data.Data_Transfer[0],0,TL70Pro.Write.General_Segment_Config.Animation_Synchro,0,2)BTD(Port_Data.Data_Transfer[1],0,TL70Pro.Write.General_Segment_Config.Background_Intensity,0,2)BTD(Port_Data.Data_Transfer[2],0,TL70Pro.Write.General_Segment_Config.Background_Color,0,2)OTU(Port_Data.Port_Read.[Port])OTL(Local_Control.6);
   24: NOP();
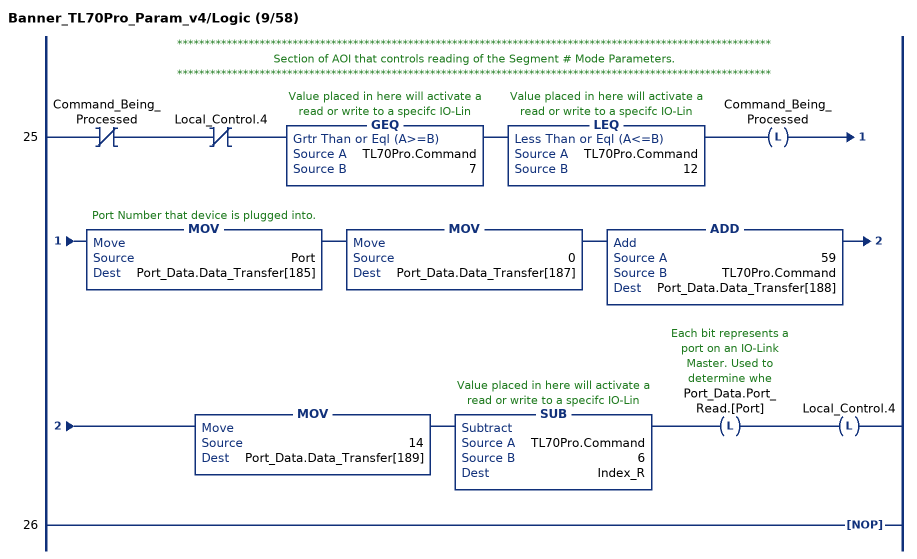
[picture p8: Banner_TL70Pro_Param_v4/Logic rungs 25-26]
   // ************************************************************************************************************
   // Section of AOI that controls reading of the Segment # Mode Parameters.
   // ************************************************************************************************************
   25: XIO(Command_Being_Processed)XIO(Local_Control.4)GEQ(TL70Pro.Command,7)LEQ(TL70Pro.Command,12)OTL(Command_Being_Processed)MOV(Port,Port_Data.Data_Transfer[185])MOV(0,Port_Data.Data_Transfer[187])ADD(59,TL70Pro.Command,Port_Data.Data_Transfer[188])MOV(14,Port_Data.Data_Transfer[189])SUB(TL70Pro.Command,6,Index_R)OTL(Port_Data.Port_Read.[Port])OTL(Local_Control.4);
   26: NOP();
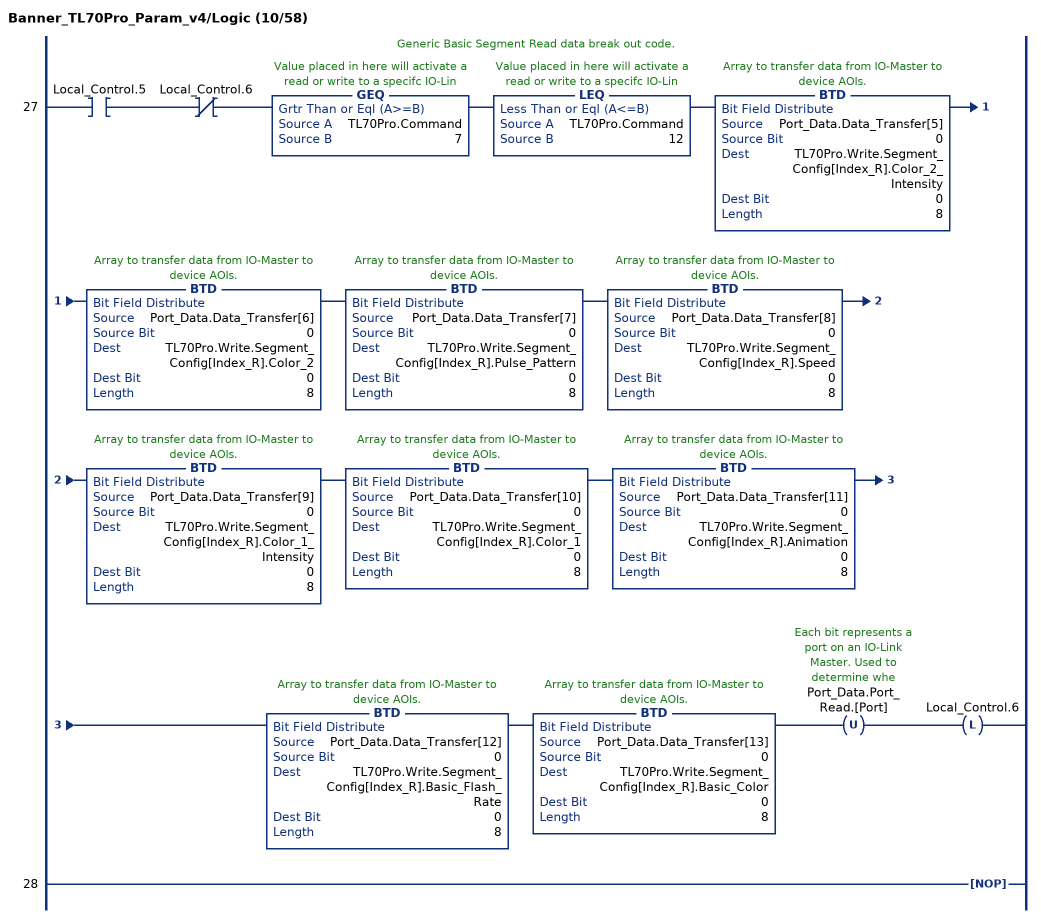
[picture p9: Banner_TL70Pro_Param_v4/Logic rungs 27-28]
   // Generic Basic Segment Read data break out code.
   27: XIC(Local_Control.5)XIO(Local_Control.6)GEQ(TL70Pro.Command,7)LEQ(TL70Pro.Command,12)BTD(Port_Data.Data_Transfer[5],0,TL70Pro.Write.Segment_Config[Index_R].Color_2_Intensity,0,8)BTD(Port_Data.Data_Transfer[6],0,TL70Pro.Write.Segment_Config[Index_R].Color_2,0,8)BTD(Port_Data.Data_Transfer[7],0,TL70Pro.Write.Segment_Config[Index_R].Pulse_Pattern,0,8)BTD(Port_Data.Data_Transfer[8],0,TL70Pro.Write.Segment_Config[Index_R].Speed,0,8)BTD(Port_Data.Data_Transfer[9],0,TL70Pro.Write.Segment_Config[Index_R].Color_1_Intensity,0,8)BTD(Port_Data.Data_Transfer[10],0,TL70Pro.Write.Segment_Config[Index_R].Color_1,0,8)BTD(Port_Data.Data_Transfer[11],0,TL70Pro.Write.Segment_Config[Index_R].Animation,0,8)BTD(Port_Data.Data_Transfer[12],0,TL70Pro.Write.Segment_Config[Index_R].Basic_Flash_Rate,0,8)BTD(Port_Data.Data_Transfer[13],0,TL70Pro.Write.Segment_Config[Index_R].Basic_Color,0,8)OTU(Port_Data.Port_Read.[Port])OTL(Local_Control.6);
   28: NOP();
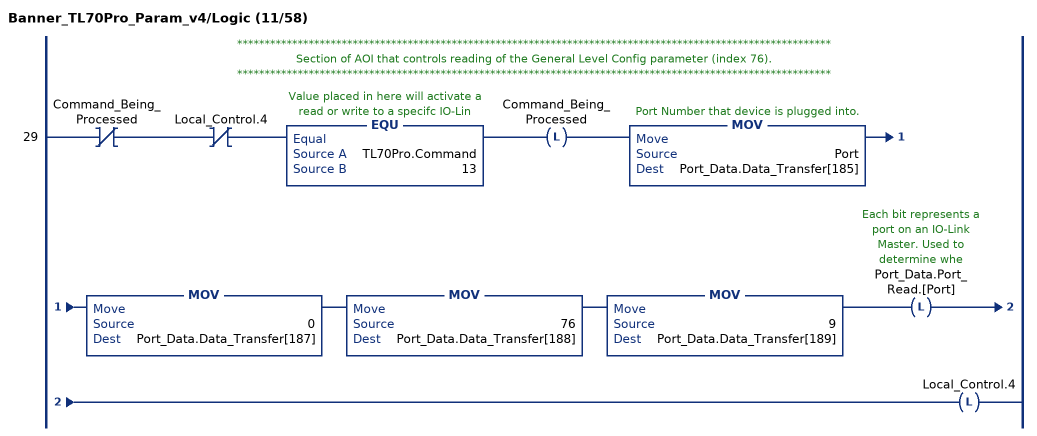
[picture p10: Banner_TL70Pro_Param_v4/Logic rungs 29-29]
   // ************************************************************************************************************
   // Section of AOI that controls reading of the General Level Config parameter (index 76).
   // ************************************************************************************************************
   29: XIO(Command_Being_Processed)XIO(Local_Control.4)EQU(TL70Pro.Command,13)OTL(Command_Being_Processed)MOV(Port,Port_Data.Data_Transfer[185])MOV(0,Port_Data.Data_Transfer[187])MOV(76,Port_Data.Data_Transfer[188])MOV(9,Port_Data.Data_Transfer[189])OTL(Port_Data.Port_Read.[Port])OTL(Local_Control.4);
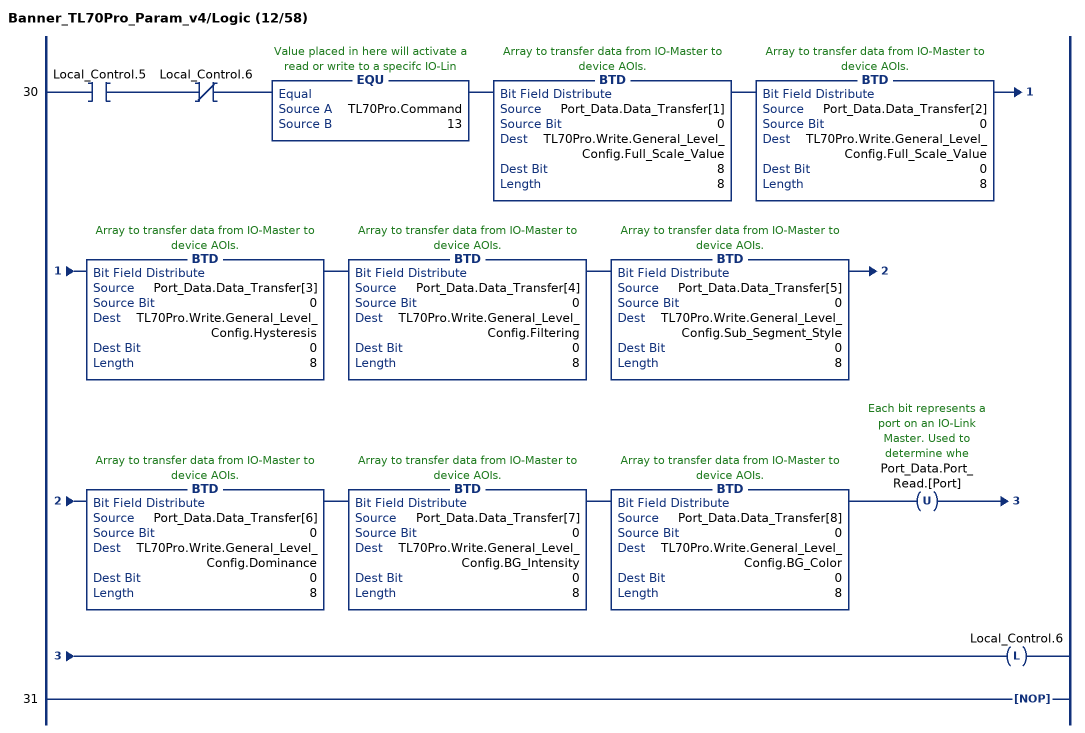
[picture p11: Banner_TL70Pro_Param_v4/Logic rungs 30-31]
   30: XIC(Local_Control.5)XIO(Local_Control.6)EQU(TL70Pro.Command,13)BTD(Port_Data.Data_Transfer[1],0,TL70Pro.Write.General_Level_Config.Full_Scale_Value,8,8)BTD(Port_Data.Data_Transfer[2],0,TL70Pro.Write.General_Level_Config.Full_Scale_Value,0,8)BTD(Port_Data.Data_Transfer[3],0,TL70Pro.Write.General_Level_Config.Hysteresis,0,8)BTD(Port_Data.Data_Transfer[4],0,TL70Pro.Write.General_Level_Config.Filtering,0,8)BTD(Port_Data.Data_Transfer[5],0,TL70Pro.Write.General_Level_Config.Sub_Segment_Style,0,8)BTD(Port_Data.Data_Transfer[6],0,TL70Pro.Write.General_Level_Config.Dominance,0,8)BTD(Port_Data.Data_Transfer[7],0,TL70Pro.Write.General_Level_Config.BG_Intensity,0,8)BTD(Port_Data.Data_Transfer[8],0,TL70Pro.Write.General_Level_Config.BG_Color,0,8)OTU(Port_Data.Port_Read.[Port])OTL(Local_Control.6);
   31: NOP();
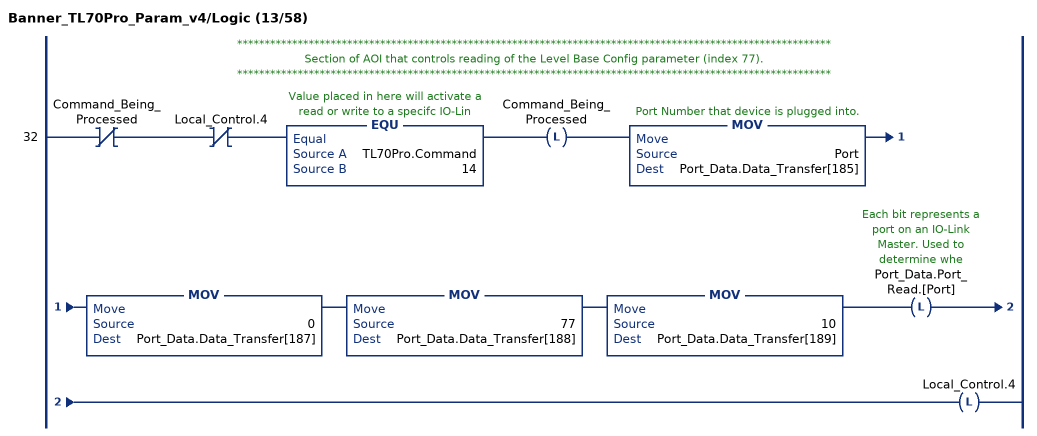
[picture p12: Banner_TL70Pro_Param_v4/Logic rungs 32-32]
   // ************************************************************************************************************
   // Section of AOI that controls reading of the Level Base Config parameter (index 77).
   // ************************************************************************************************************
   32: XIO(Command_Being_Processed)XIO(Local_Control.4)EQU(TL70Pro.Command,14)OTL(Command_Being_Processed)MOV(Port,Port_Data.Data_Transfer[185])MOV(0,Port_Data.Data_Transfer[187])MOV(77,Port_Data.Data_Transfer[188])MOV(10,Port_Data.Data_Transfer[189])OTL(Port_Data.Port_Read.[Port])OTL(Local_Control.4);
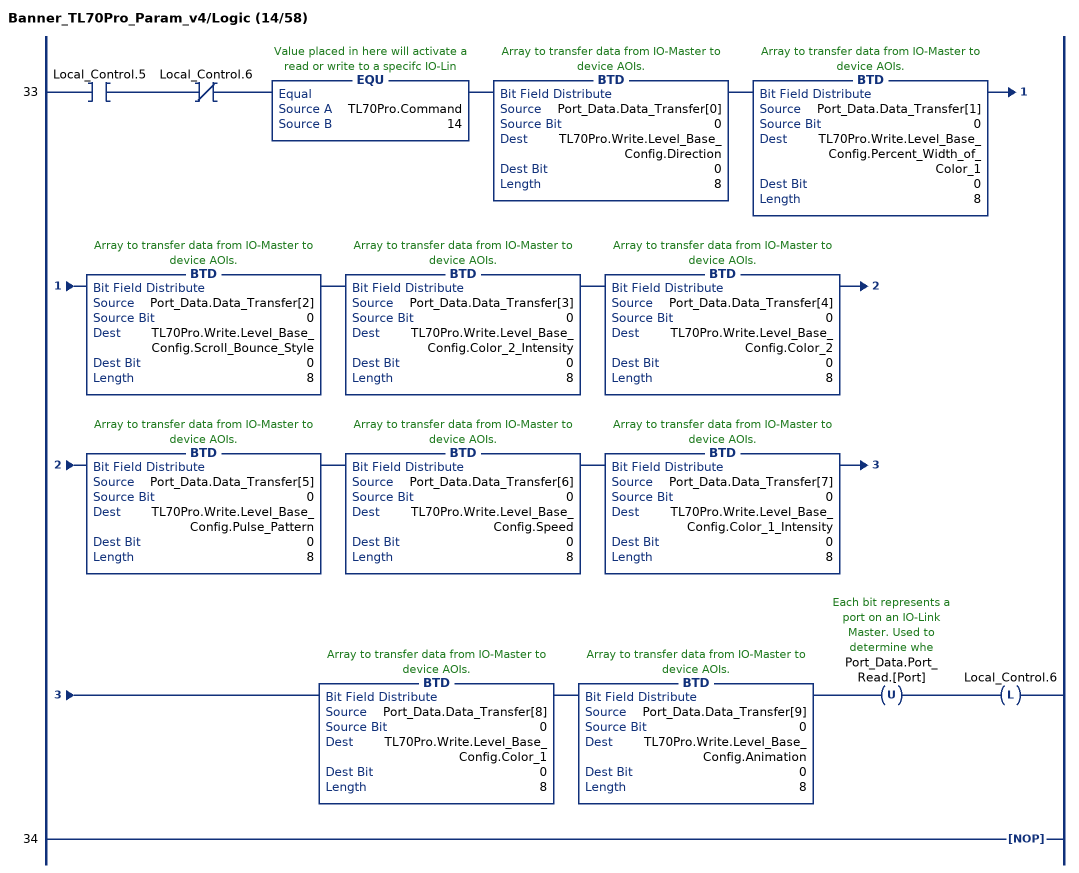
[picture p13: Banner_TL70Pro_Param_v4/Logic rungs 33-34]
   33: XIC(Local_Control.5)XIO(Local_Control.6)EQU(TL70Pro.Command,14)BTD(Port_Data.Data_Transfer[0],0,TL70Pro.Write.Level_Base_Config.Direction,0,8)BTD(Port_Data.Data_Transfer[1],0,TL70Pro.Write.Level_Base_Config.Percent_Width_of_Color_1,0,8)BTD(Port_Data.Data_Transfer[2],0,TL70Pro.Write.Level_Base_Config.Scroll_Bounce_Style,0,8)BTD(Port_Data.Data_Transfer[3],0,TL70Pro.Write.Level_Base_Config.Color_2_Intensity,0,8)BTD(Port_Data.Data_Transfer[4],0,TL70Pro.Write.Level_Base_Config.Color_2,0,8)BTD(Port_Data.Data_Transfer[5],0,TL70Pro.Write.Level_Base_Config.Pulse_Pattern,0,8)BTD(Port_Data.Data_Transfer[6],0,TL70Pro.Write.Level_Base_Config.Speed,0,8)BTD(Port_Data.Data_Transfer[7],0,TL70Pro.Write.Level_Base_Config.Color_1_Intensity,0,8)BTD(Port_Data.Data_Transfer[8],0,TL70Pro.Write.Level_Base_Config.Color_1,0,8)BTD(Port_Data.Data_Transfer[9],0,TL70Pro.Write.Level_Base_Config.Animation,0,8)OTU(Port_Data.Port_Read.[Port])OTL(Local_Control.6);
   34: NOP();
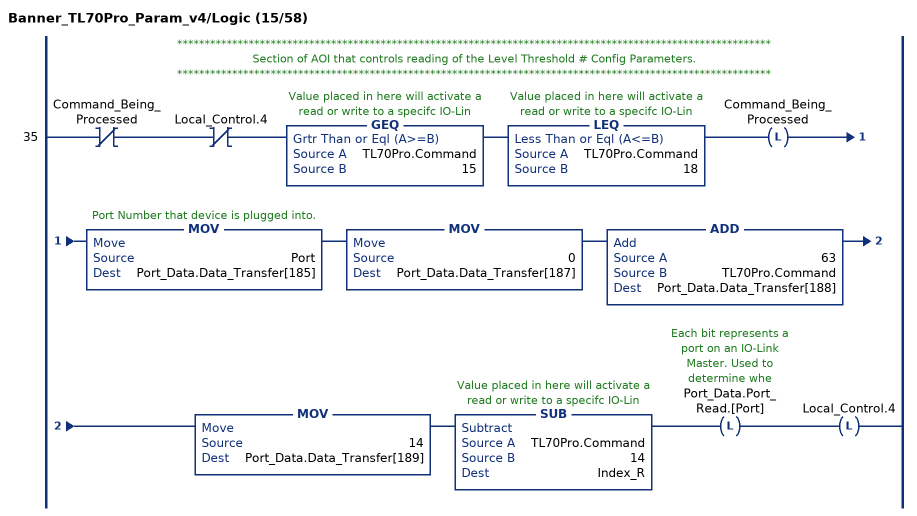
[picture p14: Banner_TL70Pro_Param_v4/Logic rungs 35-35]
   // ************************************************************************************************************
   // Section of AOI that controls reading of the Level Threshold # Config Parameters.
   // ************************************************************************************************************
   35: XIO(Command_Being_Processed)XIO(Local_Control.4)GEQ(TL70Pro.Command,15)LEQ(TL70Pro.Command,18)OTL(Command_Being_Processed)MOV(Port,Port_Data.Data_Transfer[185])MOV(0,Port_Data.Data_Transfer[187])ADD(63,TL70Pro.Command,Port_Data.Data_Transfer[188])MOV(14,Port_Data.Data_Transfer[189])SUB(TL70Pro.Command,14,Index_R)OTL(Port_Data.Port_Read.[Port])OTL(Local_Control.4);
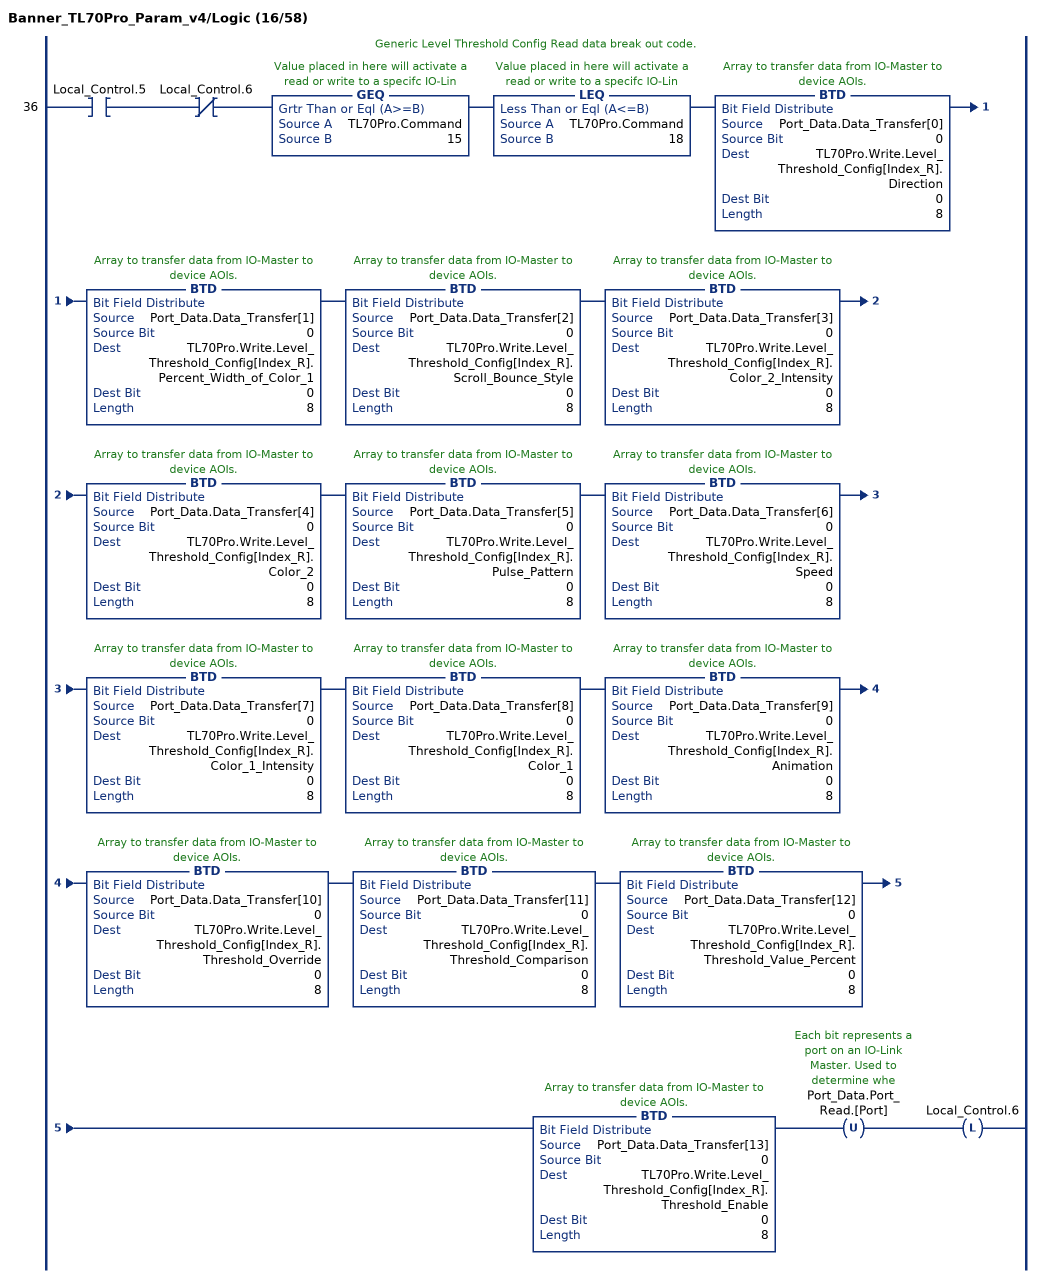
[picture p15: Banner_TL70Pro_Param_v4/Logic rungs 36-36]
   // Generic Level Threshold Config Read data break out code.
   36: XIC(Local_Control.5)XIO(Local_Control.6)GEQ(TL70Pro.Command,15)LEQ(TL70Pro.Command,18)BTD(Port_Data.Data_Transfer[0],0,TL70Pro.Write.Level_Threshold_Config[Index_R].Direction,0,8)BTD(Port_Data.Data_Transfer[1],0,TL70Pro.Write.Level_Threshold_Config[Index_R].Percent_Width_of_Color_1,0,8)BTD(Port_Data.Data_Transfer[2],0,TL70Pro.Write.Level_Threshold_Config[Index_R].Scroll_Bounce_Style,0,8)BTD(Port_Data.Data_Transfer[3],0,TL70Pro.Write.Level_Threshold_Config[Index_R].Color_2_Intensity,0,8)BTD(Port_Data.Data_Transfer[4],0,TL70Pro.Write.Level_Threshold_Config[Index_R].Color_2,0,8)BTD(Port_Data.Data_Transfer[5],0,TL70Pro.Write.Level_Threshold_Config[Index_R].Pulse_Pattern,0,8)BTD(Port_Data.Data_Transfer[6],0,TL70Pro.Write.Level_Threshold_Config[Index_R].Speed,0,8)BTD(Port_Data.Data_Transfer[7],0,TL70Pro.Write.Level_Threshold_Config[Index_R].Color_1_Intensity,0,8)BTD(Port_Data.Data_Transfer[8],0,TL70Pro.Write.Level_Threshold_Config[Index_R].Color_1,0,8)BTD(Port_Data.Data_Transfer[9],0,TL70Pro.Write.Level_Threshold_Config[Index_R].Animation,0,8)BTD(Port_Data.Data_Transfer[10],0,TL70Pro.Write.Level_Threshold_Config[Index_R].Threshold_Override,0,8)BTD(Port_Data.Data_Transfer[11],0,TL70Pro.Write.Level_Threshold_Config[Index_R].Threshold_Comparison,0,8)BTD(Port_Data.Data_Transfer[12],0,TL70Pro.Write.Level_Threshold_Config[Index_R].Threshold_Value_Percent,0,8)BTD(Port_Data.Data_Transfer[13],0,TL70Pro.Write.Level_Threshold_Config[Index_R].Threshold_Enable,0,8)OTU(Port_Data.Port_Read.[Port])OTL(Local_Control.6);
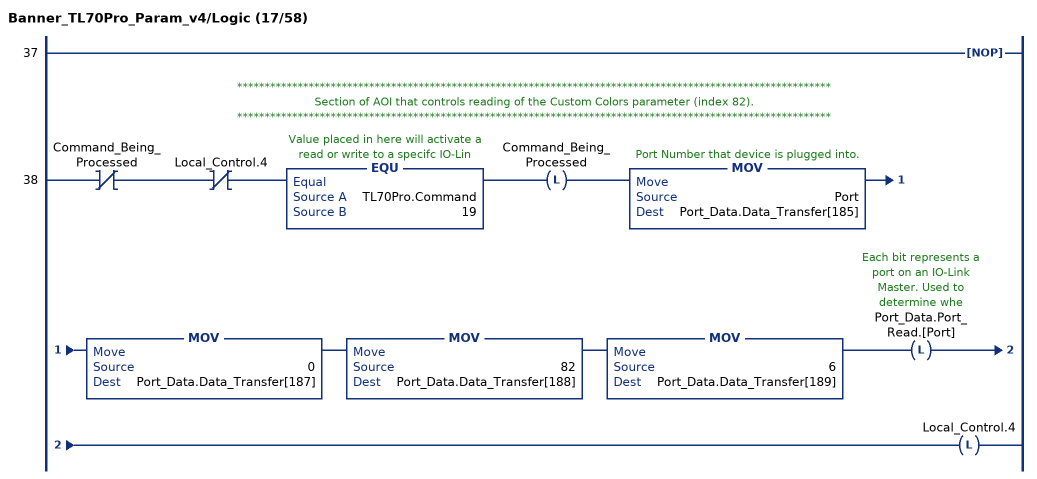
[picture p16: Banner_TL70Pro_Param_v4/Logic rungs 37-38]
   37: NOP();
   // ************************************************************************************************************
   // Section of AOI that controls reading of the Custom Colors parameter (index 82).
   // ************************************************************************************************************
   38: XIO(Command_Being_Processed)XIO(Local_Control.4)EQU(TL70Pro.Command,19)OTL(Command_Being_Processed)MOV(Port,Port_Data.Data_Transfer[185])MOV(0,Port_Data.Data_Transfer[187])MOV(82,Port_Data.Data_Transfer[188])MOV(6,Port_Data.Data_Transfer[189])OTL(Port_Data.Port_Read.[Port])OTL(Local_Control.4);
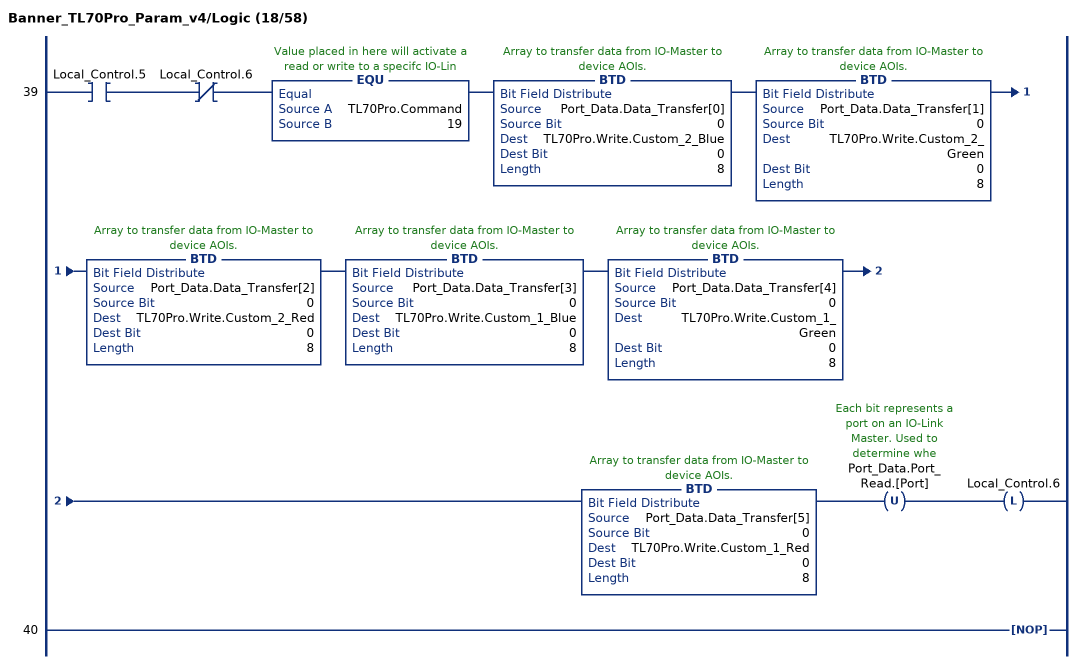
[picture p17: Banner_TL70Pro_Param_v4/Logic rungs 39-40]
   39: XIC(Local_Control.5)XIO(Local_Control.6)EQU(TL70Pro.Command,19)BTD(Port_Data.Data_Transfer[0],0,TL70Pro.Write.Custom_2_Blue,0,8)BTD(Port_Data.Data_Transfer[1],0,TL70Pro.Write.Custom_2_Green,0,8)BTD(Port_Data.Data_Transfer[2],0,TL70Pro.Write.Custom_2_Red,0,8)BTD(Port_Data.Data_Transfer[3],0,TL70Pro.Write.Custom_1_Blue,0,8)BTD(Port_Data.Data_Transfer[4],0,TL70Pro.Write.Custom_1_Green,0,8)BTD(Port_Data.Data_Transfer[5],0,TL70Pro.Write.Custom_1_Red,0,8)OTU(Port_Data.Port_Read.[Port])OTL(Local_Control.6);
   40: NOP();
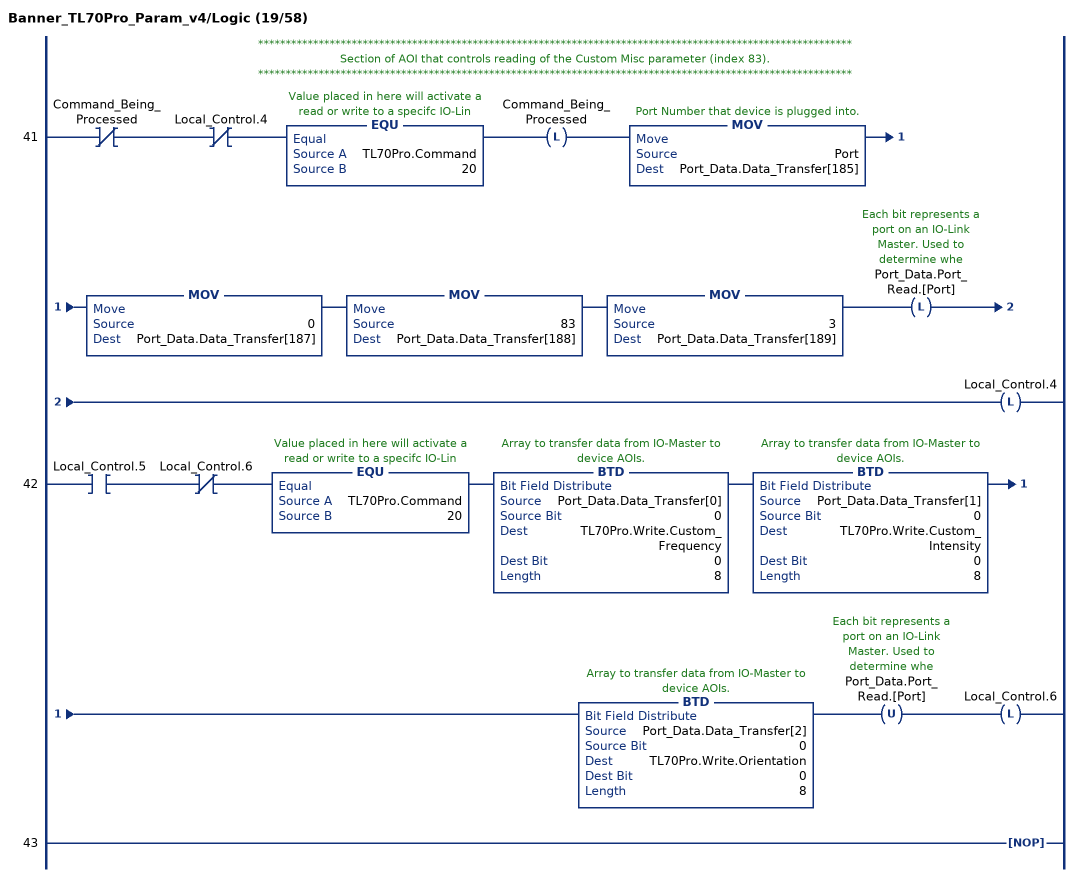
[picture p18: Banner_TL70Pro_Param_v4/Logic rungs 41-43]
   // ************************************************************************************************************
   // Section of AOI that controls reading of the Custom Misc parameter (index 83).
   // ************************************************************************************************************
   41: XIO(Command_Being_Processed)XIO(Local_Control.4)EQU(TL70Pro.Command,20)OTL(Command_Being_Processed)MOV(Port,Port_Data.Data_Transfer[185])MOV(0,Port_Data.Data_Transfer[187])MOV(83,Port_Data.Data_Transfer[188])MOV(3,Port_Data.Data_Transfer[189])OTL(Port_Data.Port_Read.[Port])OTL(Local_Control.4);
   42: XIC(Local_Control.5)XIO(Local_Control.6)EQU(TL70Pro.Command,20)BTD(Port_Data.Data_Transfer[0],0,TL70Pro.Write.Custom_Frequency,0,8)BTD(Port_Data.Data_Transfer[1],0,TL70Pro.Write.Custom_Intensity,0,8)BTD(Port_Data.Data_Transfer[2],0,TL70Pro.Write.Orientation,0,8)OTU(Port_Data.Port_Read.[Port])OTL(Local_Control.6);
   43: NOP();
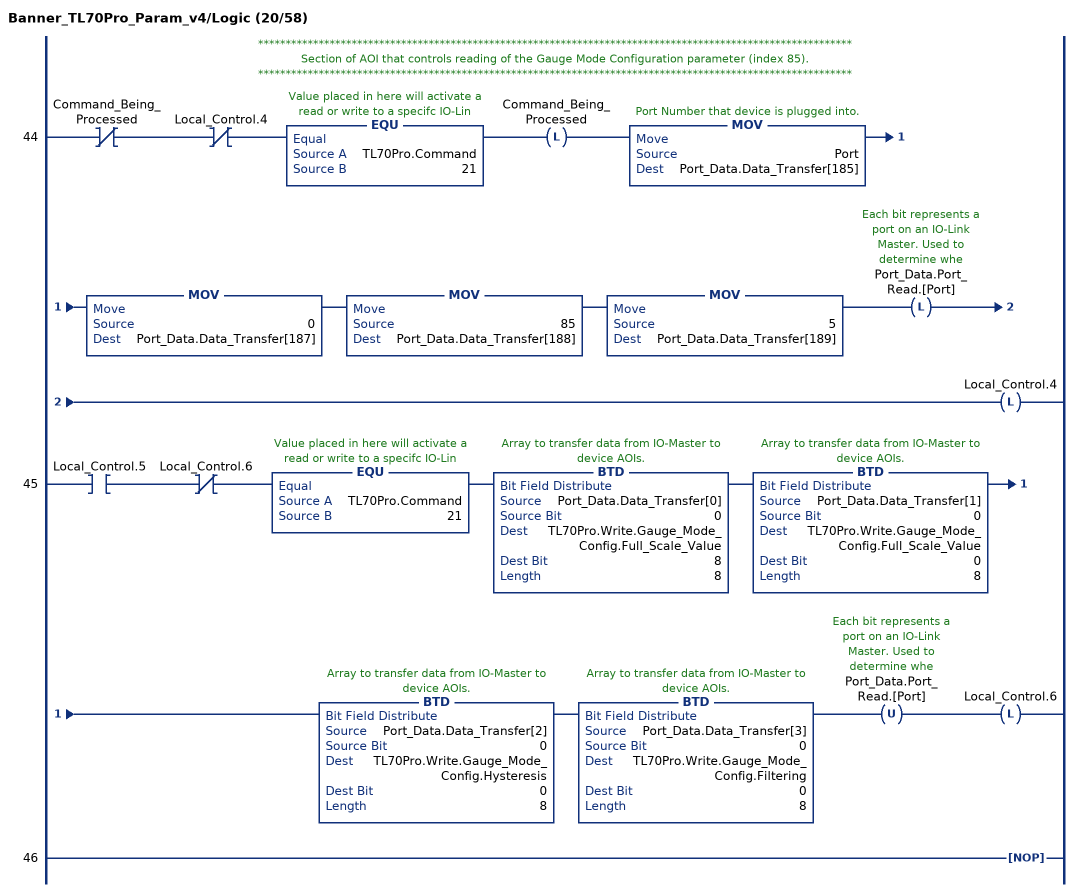
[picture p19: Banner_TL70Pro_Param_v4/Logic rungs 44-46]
   // ************************************************************************************************************
   // Section of AOI that controls reading of the Gauge Mode Configuration parameter (index 85).
   // ************************************************************************************************************
   44: XIO(Command_Being_Processed)XIO(Local_Control.4)EQU(TL70Pro.Command,21)OTL(Command_Being_Processed)MOV(Port,Port_Data.Data_Transfer[185])MOV(0,Port_Data.Data_Transfer[187])MOV(85,Port_Data.Data_Transfer[188])MOV(5,Port_Data.Data_Transfer[189])OTL(Port_Data.Port_Read.[Port])OTL(Local_Control.4);
   45: XIC(Local_Control.5)XIO(Local_Control.6)EQU(TL70Pro.Command,21)BTD(Port_Data.Data_Transfer[0],0,TL70Pro.Write.Gauge_Mode_Config.Full_Scale_Value,8,8)BTD(Port_Data.Data_Transfer[1],0,TL70Pro.Write.Gauge_Mode_Config.Full_Scale_Value,0,8)BTD(Port_Data.Data_Transfer[2],0,TL70Pro.Write.Gauge_Mode_Config.Hysteresis,0,8)BTD(Port_Data.Data_Transfer[3],0,TL70Pro.Write.Gauge_Mode_Config.Filtering,0,8)OTU(Port_Data.Port_Read.[Port])OTL(Local_Control.6);
   46: NOP();
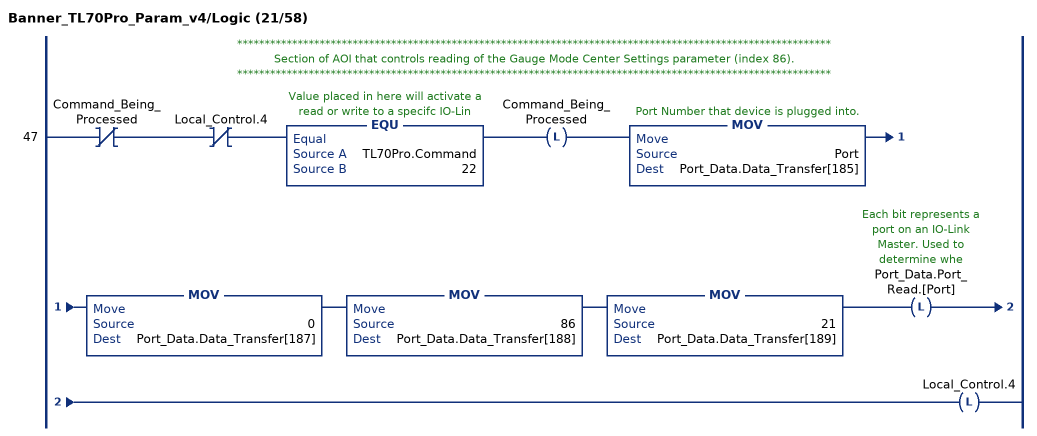
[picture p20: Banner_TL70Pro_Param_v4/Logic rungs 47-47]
   // ************************************************************************************************************
   // Section of AOI that controls reading of the Gauge Mode Center Settings parameter (index 86).
   // ************************************************************************************************************
   47: XIO(Command_Being_Processed)XIO(Local_Control.4)EQU(TL70Pro.Command,22)OTL(Command_Being_Processed)MOV(Port,Port_Data.Data_Transfer[185])MOV(0,Port_Data.Data_Transfer[187])MOV(86,Port_Data.Data_Transfer[188])MOV(21,Port_Data.Data_Transfer[189])OTL(Port_Data.Port_Read.[Port])OTL(Local_Control.4);
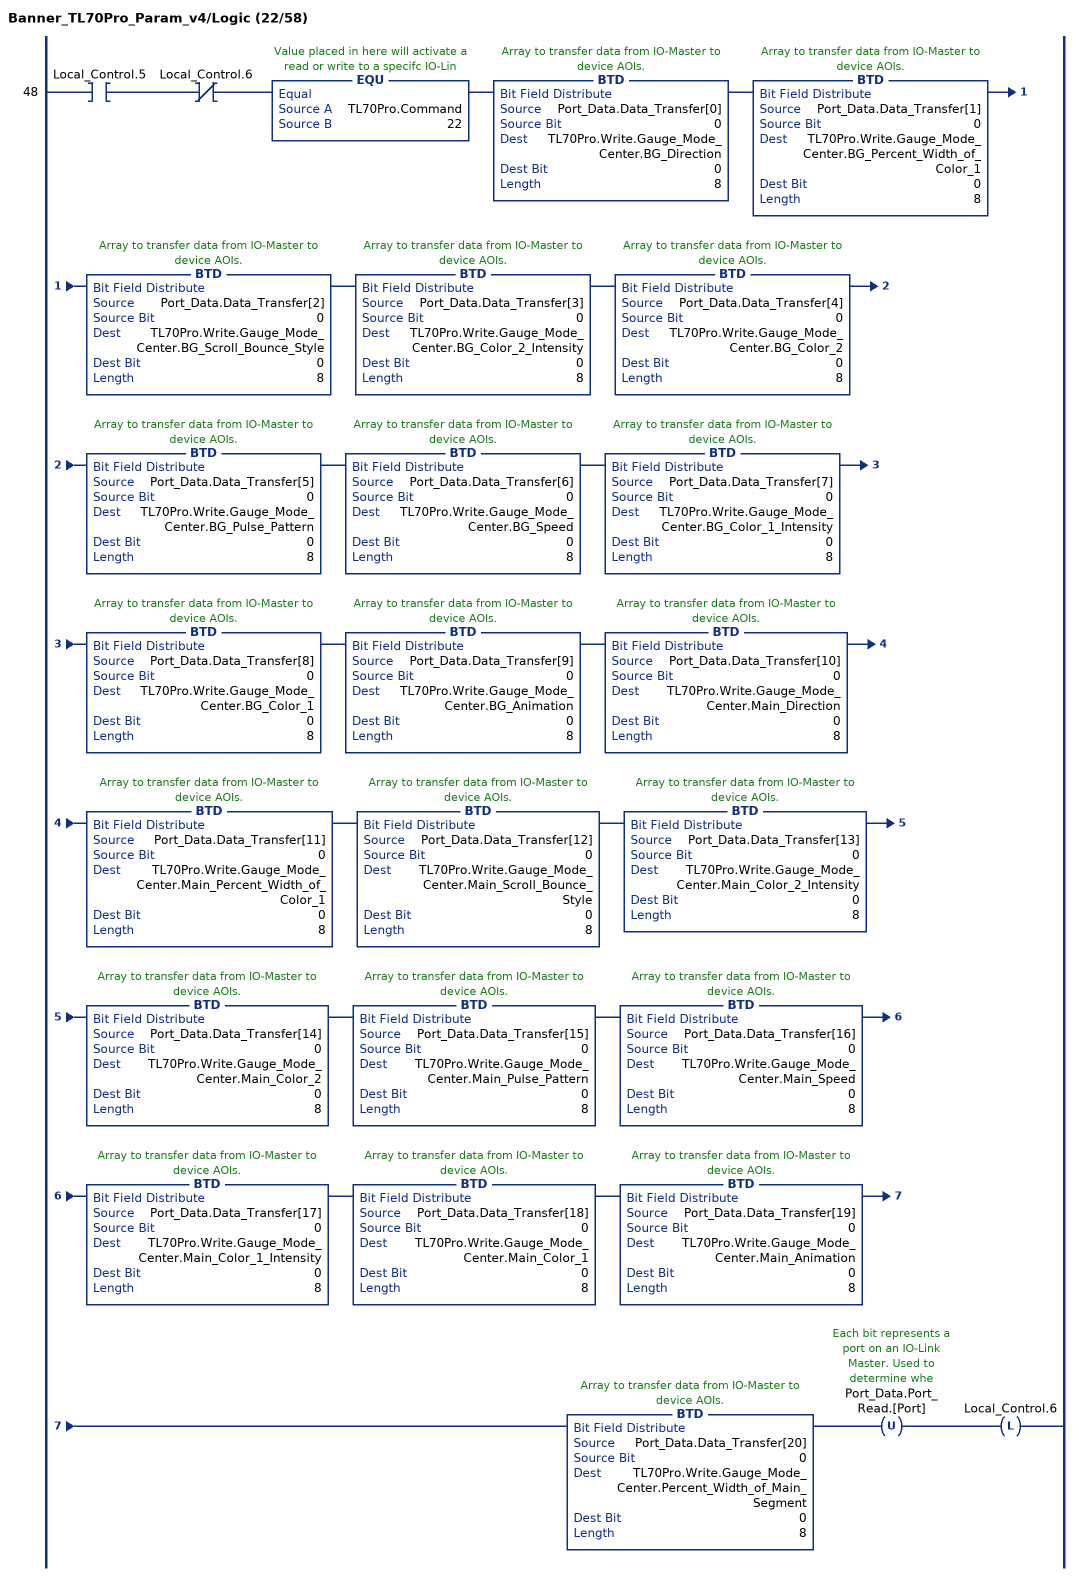
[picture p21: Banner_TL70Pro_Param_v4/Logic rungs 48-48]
   48: XIC(Local_Control.5)XIO(Local_Control.6)EQU(TL70Pro.Command,22)BTD(Port_Data.Data_Transfer[0],0,TL70Pro.Write.Gauge_Mode_Center.BG_Direction,0,8)BTD(Port_Data.Data_Transfer[1],0,TL70Pro.Write.Gauge_Mode_Center.BG_Percent_Width_of_Color_1,0,8)BTD(Port_Data.Data_Transfer[2],0,TL70Pro.Write.Gauge_Mode_Center.BG_Scroll_Bounce_Style,0,8)BTD(Port_Data.Data_Transfer[3],0,TL70Pro.Write.Gauge_Mode_Center.BG_Color_2_Intensity,0,8)BTD(Port_Data.Data_Transfer[4],0,TL70Pro.Write.Gauge_Mode_Center.BG_Color_2,0,8)BTD(Port_Data.Data_Transfer[5],0,TL70Pro.Write.Gauge_Mode_Center.BG_Pulse_Pattern,0,8)BTD(Port_Data.Data_Transfer[6],0,TL70Pro.Write.Gauge_Mode_Center.BG_Speed,0,8)BTD(Port_Data.Data_Transfer[7],0,TL70Pro.Write.Gauge_Mode_Center.BG_Color_1_Intensity,0,8)BTD(Port_Data.Data_Transfer[8],0,TL70Pro.Write.Gauge_Mode_Center.BG_Color_1,0,8)BTD(Port_Data.Data_Transfer[9],0,TL70Pro.Write.Gauge_Mode_Center.BG_Animation,0,8)BTD(Port_Data.Data_Transfer[10],0,TL70Pro.Write.Gauge_Mode_Center.Main_Direction,0,8)BTD(Port_Data.Data_Transfer[11],0,TL70Pro.Write.Gauge_Mode_Center.Main_Percent_Width_of_Color_1,0,8)BTD(Port_Data.Data_Transfer[12],0,TL70Pro.Write.Gauge_Mode_Center.Main_Scroll_Bounce_Style,0,8)BTD(Port_Data.Data_Transfer[13],0,TL70Pro.Write.Gauge_Mode_Center.Main_Color_2_Intensity,0,8)BTD(Port_Data.Data_Transfer[14],0,TL70Pro.Write.Gauge_Mode_Center.Main_Color_2,0,8)BTD(Port_Data.Data_Transfer[15],0,TL70Pro.Write.Gauge_Mode_Center.Main_Pulse_Pattern,0,8)BTD(Port_Data.Data_Transfer[16],0,TL70Pro.Write.Gauge_Mode_Center.Main_Speed,0,8)BTD(Port_Data.Data_Transfer[17],0,TL70Pro.Write.Gauge_Mode_Center.Main_Color_1_Intensity,0,8)BTD(Port_Data.Data_Transfer[18],0,TL70Pro.Write.Gauge_Mode_Center.Main_Color_1,0,8)BTD(Port_Data.Data_Transfer[19],0,TL70Pro.Write.Gauge_Mode_Center.Main_Animation,0,8)BTD(Port_Data.Data_Transfer[20],0,TL70Pro.Write.Gauge_Mode_Center.Percent_Width_of_Main_Segment,0,8)OTU(Port_Data.Port_Read.[Port])OTL(Local_Control.6);
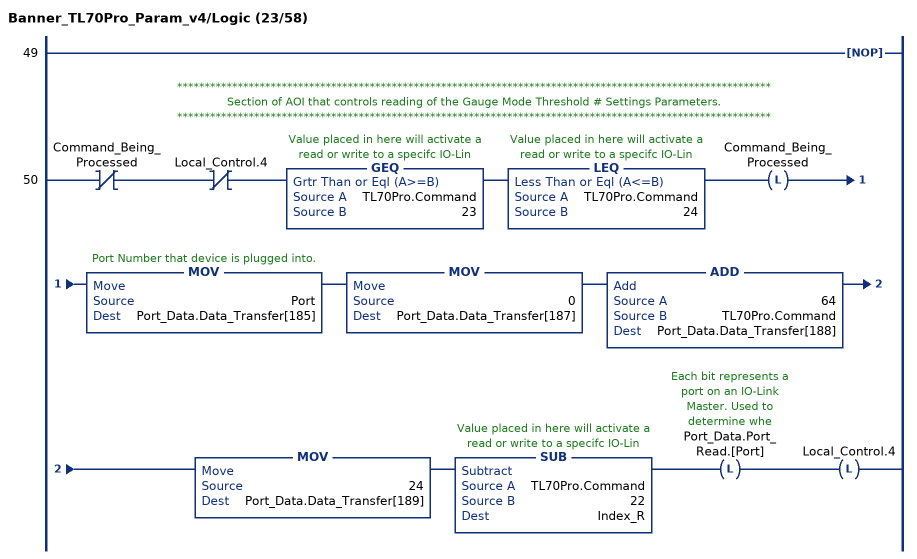
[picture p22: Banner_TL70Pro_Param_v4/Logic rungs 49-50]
   49: NOP();
   // ************************************************************************************************************
   // Section of AOI that controls reading of the Gauge Mode Threshold # Settings Parameters.
   // ************************************************************************************************************
   50: XIO(Command_Being_Processed)XIO(Local_Control.4)GEQ(TL70Pro.Command,23)LEQ(TL70Pro.Command,24)OTL(Command_Being_Processed)MOV(Port,Port_Data.Data_Transfer[185])MOV(0,Port_Data.Data_Transfer[187])ADD(64,TL70Pro.Command,Port_Data.Data_Transfer[188])MOV(24,Port_Data.Data_Transfer[189])SUB(TL70Pro.Command,22,Index_R)OTL(Port_Data.Port_Read.[Port])OTL(Local_Control.4);
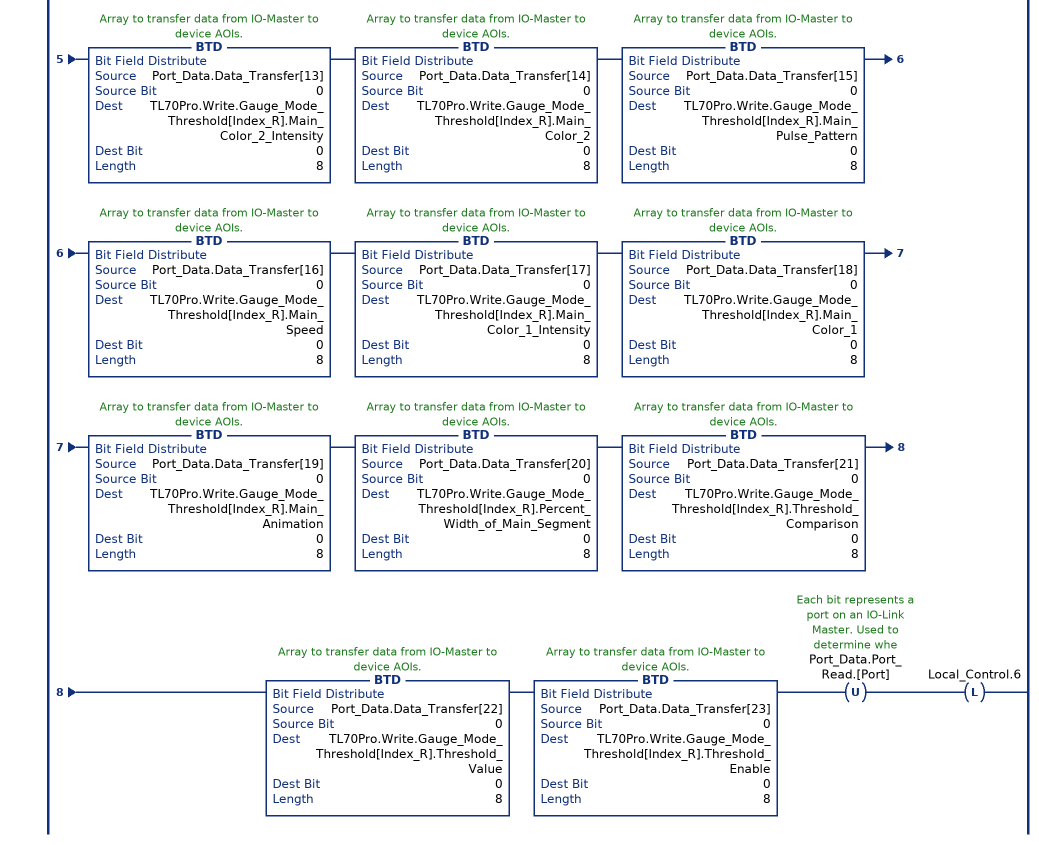
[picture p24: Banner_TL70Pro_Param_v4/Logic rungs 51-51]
   // Generic Gauge Mode # Threshold Read data break out code.
   51: XIC(Local_Control.5)XIO(Local_Control.6)GEQ(TL70Pro.Command,23)LEQ(TL70Pro.Command,24)BTD(Port_Data.Data_Transfer[0],0,TL70Pro.Write.Gauge_Mode_Threshold[Index_R].BG_Direction,0,8)BTD(Port_Data.Data_Transfer[1],0,TL70Pro.Write.Gauge_Mode_Threshold[Index_R].BG_Percent_Width_of_Color_1,0,8)BTD(Port_Data.Data_Transfer[2],0,TL70Pro.Write.Gauge_Mode_Threshold[Index_R].BG_Scroll_Bounce_Style,0,8)BTD(Port_Data.Data_Transfer[3],0,TL70Pro.Write.Gauge_Mode_Threshold[Index_R].BG_Color_2_Intensity,0,8)BTD(Port_Data.Data_Transfer[4],0,TL70Pro.Write.Gauge_Mode_Threshold[Index_R].BG_Color_2,0,8)BTD(Port_Data.Data_Transfer[5],0,TL70Pro.Write.Gauge_Mode_Threshold[Index_R].BG_Pulse_Pattern,0,8)BTD(Port_Data.Data_Transfer[6],0,TL70Pro.Write.Gauge_Mode_Threshold[Index_R].BG_Speed,0,8)BTD(Port_Data.Data_Transfer[7],0,TL70Pro.Write.Gauge_Mode_Threshold[Index_R].BG_Color_1_Intensity,0,8)BTD(Port_Data.Data_Transfer[8],0,TL70Pro.Write.Gauge_Mode_Threshold[Index_R].BG_Color_1,0,8)BTD(Port_Data.Data_Transfer[9],0,TL70Pro.Write.Gauge_Mode_Threshold[Index_R].BG_Animation,0,8)BTD(Port_Data.Data_Transfer[10],0,TL70Pro.Write.Gauge_Mode_Threshold[Index_R].Main_Direction,0,8)BTD(Port_Data.Data_Transfer[11],0,TL70Pro.Write.Gauge_Mode_Threshold[Index_R].Main_Percent_Width_of_Color_1,0,8)BTD(Port_Data.Data_Transfer[12],0,TL70Pro.Write.Gauge_Mode_Threshold[Index_R].Main_Scroll_Bounce_Style,0,8)BTD(Port_Data.Data_Transfer[13],0,TL70Pro.Write.Gauge_Mode_Threshold[Index_R].Main_Color_2_Intensity,0,8)BTD(Port_Data.Data_Transfer[14],0,TL70Pro.Write.Gauge_Mode_Threshold[Index_R].Main_Color_2,0,8)BTD(Port_Data.Data_Transfer[15],0,TL70Pro.Write.Gauge_Mode_Threshold[Index_R].Main_Pulse_Pattern,0,8)BTD(Port_Data.Data_Transfer[16],0,TL70Pro.Write.Gauge_Mode_Threshold[Index_R].Main_Speed,0,8)BTD(Port_Data.Data_Transfer[17],0,TL70Pro.Write.Gauge_Mode_Threshold[Index_R].Main_Color_1_Intensity,0,8)BTD(Port_Data.Data_Transfer[18],0,TL70Pro.Write.Gauge_Mode_Threshold[Index_R].Main_Color_1,0,8)BTD(Port_Data.Data_Transfer[19],0,TL70Pro.Write.Gauge_Mode_Threshold[Index_R].Main_Animation,0,8)BTD(Port_Data.Data_Transfer[20],0,TL70Pro.Write.Gauge_Mode_Threshold[Index_R].Percent_Width_of_Main_Segment,0,8)BTD(Port_Data.Data_Transfer[21],0,TL70Pro.Write.Gauge_Mode_Threshold[Index_R].Threshold_Comparison,0,8)BTD(Port_Data.Data_Transfer[22],0,TL70Pro.Write.Gauge_Mode_Threshold[Index_R].Threshold_Value,0,8)BTD(Port_Data.Data_Transfer[23],0,TL70Pro.Write.Gauge_Mode_Threshold[Index_R].Threshold_Enable,0,8)OTU(Port_Data.Port_Read.[Port])OTL(Local_Control.6);
